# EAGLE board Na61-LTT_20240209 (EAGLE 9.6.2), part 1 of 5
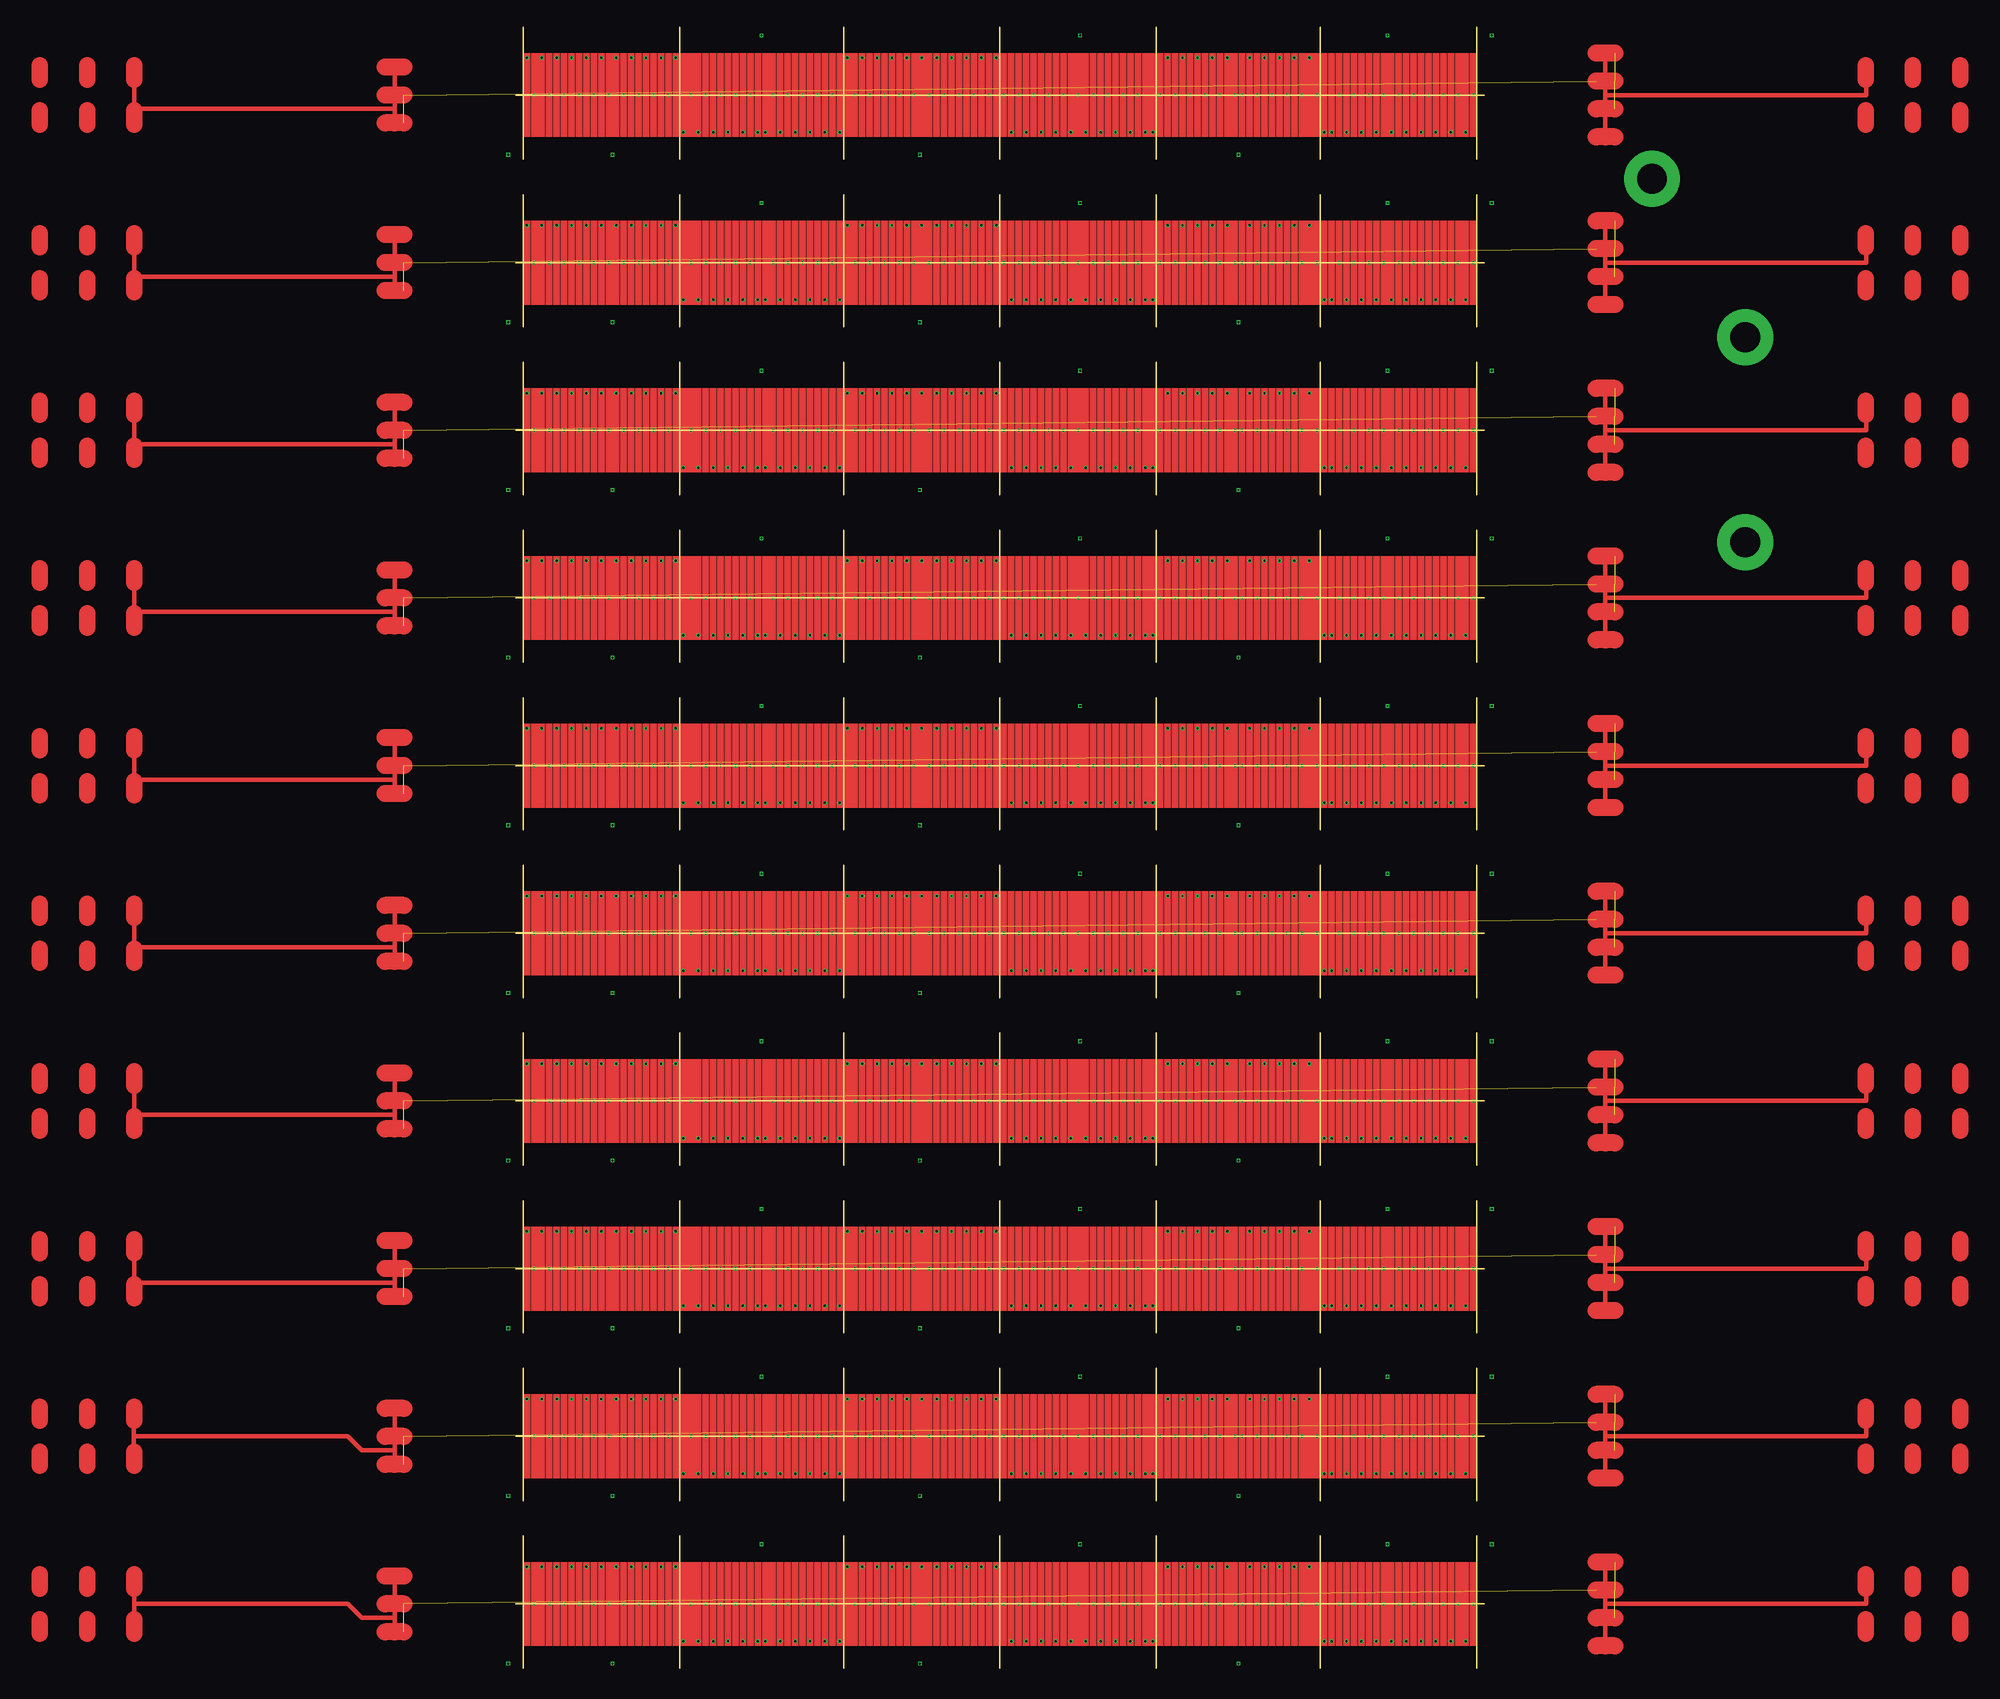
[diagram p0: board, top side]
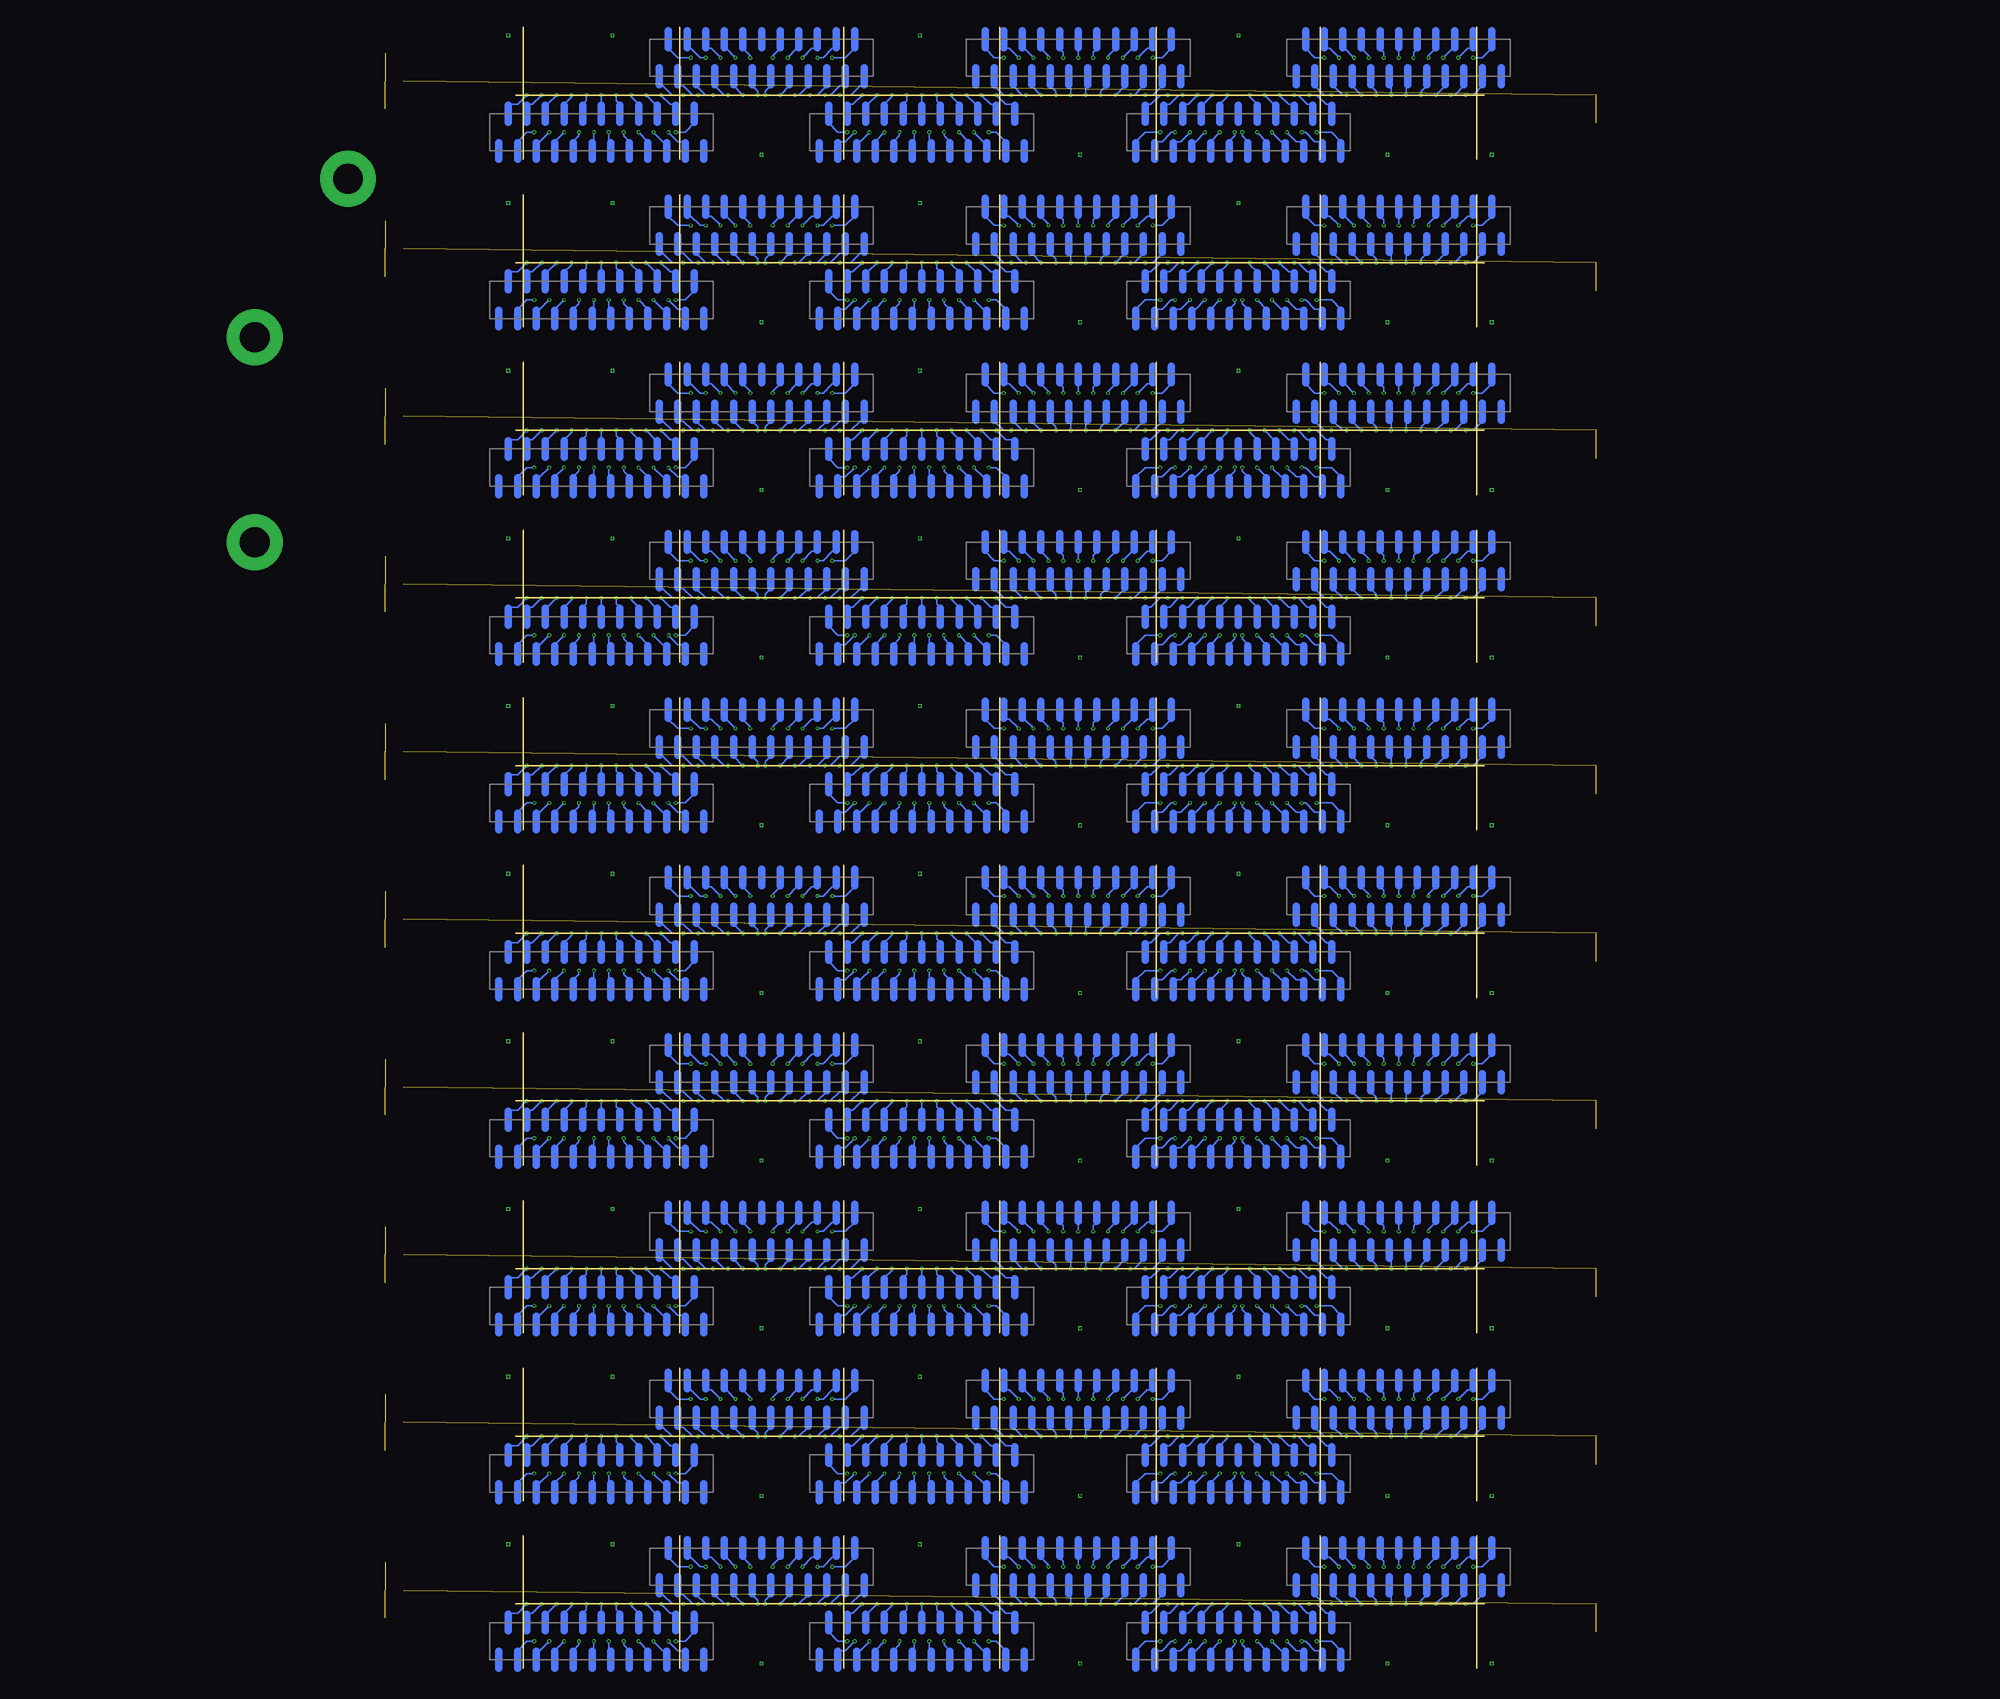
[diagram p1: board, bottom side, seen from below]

Size 104 x 176.2 mm. Coordinates in mm from the lower left corner, seen from the top.
Outline: 80 segments
Copper layers (1*16): Top 0.035mm / dielectric 1.5mm / Bottom 0.035mm
Design rules "default *": minimum track width 6mil, minimum drill 0.2mm, track to track 6mil, track to pad 6mil, pad to pad 6mil, via to via 6mil, smd to smd 6mil, copper to edge 40mil, drill to drill 6mil, minimum pad ring 8mil, minimum via ring 4mil, stop-mask expansion 4mil, vias tented up to drill 0mil, thermal gap 10mil

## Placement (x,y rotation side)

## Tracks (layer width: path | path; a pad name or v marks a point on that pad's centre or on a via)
S$1
  Bottom 0.8: 63.4,1.8 63.4,0
S$2
  Bottom 0.8: 62.4,4 62.4,5.8
S$3
  Bottom 0.8: 59.4,1.8 59.4,0
S$4
  Bottom 0.8: 56.4,4 56.4,5.8
S$5
  Bottom 0.8: 53.4,1.8 53.4,0
S$6
  Bottom 0.8: 52.4,4 52.4,5.8
S$7
  Bottom 0.8: 49.4,1.8 49.4,0
S$8
  Bottom 0.8: 50.4,4 50.4,5.8
S$9
  Bottom 0.8: 71.4,1.8 71.4,0
S$10
  Bottom 0.8: 70.4,4 70.4,5.8
S$11
  Bottom 0.8: 67.4,1.8 67.4,0
S$12
  Bottom 0.8: 66.4,4 66.4,5.8
S$13
  Bottom 0.8: 68.4,4 68.4,5.8
S$14
  Bottom 0.8: 69.4,1.8 69.4,0
S$15
  Bottom 0.8: 65.4,1.8 65.4,0
S$16
  Bottom 0.8: 64.4,4 64.4,5.8
S$17
  Bottom 0.8: 60.4,4 60.4,5.8
S$18
  Bottom 0.8: 61.4,1.8 61.4,0
S$19
  Bottom 0.8: 57.4,1.8 57.4,0
S$20
  Bottom 0.8: 58.4,4 58.4,5.8
S$21
  Bottom 0.8: 54.4,4 54.4,5.8
S$22
  Bottom 0.8: 55.4,1.8 55.4,0
S$23
  Bottom 0.8: 51.4,1.8 51.4,0
S$24
  Bottom 0.8: 44.6,9.8 44.6,8
S$25
  Bottom 0.8: 46.6,9.8 46.6,8
S$26
  Bottom 0.8: 43.6,12 43.6,13.8
S$27
  Bottom 0.8: 45.6,12 45.6,13.8
S$28
  Bottom 0.8: 40.6,9.8 40.6,8
S$29
  Bottom 0.8: 42.6,9.8 42.6,8
S$30
  Bottom 0.8: 41.6,12 41.6,13.8
S$31
  Bottom 0.8: 39.6,12 39.6,13.8
S$32
  Bottom 0.8: 38.6,9.8 38.6,8
S$33
  Bottom 0.8: 36.6,9.8 36.6,8
S$34
  Bottom 0.8: 37.6,12 37.6,13.8
S$35
  Bottom 0.8: 35.6,12 35.6,13.8
S$36
  Bottom 0.8: 34.6,9.8 34.6,8
S$37
  Bottom 0.8: 32.6,9.8 32.6,8
S$38
  Bottom 0.8: 33.6,12 33.6,13.8
S$39
  Bottom 0.8: 52.6,9.8 52.6,8
S$40
  Bottom 0.8: 54.6,9.8 54.6,8
S$41
  Bottom 0.8: 51.6,12 51.6,13.8
S$42
  Bottom 0.8: 53.6,12 53.6,13.8
S$43
  Bottom 0.8: 48.6,9.8 48.6,8
S$44
  Bottom 0.8: 50.6,9.8 50.6,8
S$45
  Bottom 0.8: 47.6,12 47.6,13.8
S$46
  Bottom 0.8: 49.6,12 49.6,13.8
S$47
  Bottom 0.8: 27.4,1.8 27.4,0
S$48
  Bottom 0.8: 29.4,1.8 29.4,0
S$49
  Bottom 0.8: 26.4,4 26.4,5.8
S$50
  Bottom 0.8: 28.4,4 28.4,5.8
S$51
  Bottom 0.8: 23.4,1.8 23.4,0
S$52
  Bottom 0.8: 25.4,1.8 25.4,0
S$53
  Bottom 0.8: 24.4,4 24.4,5.8
S$54
  Bottom 0.8: 22.4,4 22.4,5.8
S$55
  Bottom 0.8: 21.4,1.8 21.4,0
S$56
  Bottom 0.8: 19.4,1.8 19.4,0
S$57
  Bottom 0.8: 20.4,4 20.4,5.8
S$58
  Bottom 0.8: 18.4,4 18.4,5.8
S$59
  Bottom 0.8: 17.4,1.8 17.4,0
S$60
  Bottom 0.8: 15.4,1.8 15.4,0
S$61
  Bottom 0.8: 16.4,4 16.4,5.8
S$62
  Bottom 0.8: 35.4,1.8 35.4,0
S$63
  Bottom 0.8: 37.4,1.8 37.4,0
S$64
  Bottom 0.8: 34.4,4 34.4,5.8
S$65
  Bottom 0.8: 36.4,4 36.4,5.8
S$66
  Bottom 0.8: 31.4,1.8 31.4,0
S$67
  Bottom 0.8: 33.4,1.8 33.4,0
S$68
  Bottom 0.8: 30.4,4 30.4,5.8
S$69
  Bottom 0.8: 32.4,4 32.4,5.8
S$70
  Bottom 0.8: 78.6,9.8 78.6,8
S$71
  Bottom 0.8: 80.6,9.8 80.6,8
S$72
  Bottom 0.8: 77.6,12 77.6,13.8
S$73
  Bottom 0.8: 79.6,12 79.6,13.8
S$74
  Bottom 0.8: 74.6,9.8 74.6,8
S$75
  Bottom 0.8: 76.6,9.8 76.6,8
S$76
  Bottom 0.8: 75.6,12 75.6,13.8
S$77
  Bottom 0.8: 73.6,12 73.6,13.8
S$78
  Bottom 0.8: 72.6,9.8 72.6,8
S$79
  Bottom 0.8: 70.6,9.8 70.6,8
S$80
  Bottom 0.8: 71.6,12 71.6,13.8
S$81
  Bottom 0.8: 69.6,12 69.6,13.8
S$82
  Bottom 0.8: 68.6,9.8 68.6,8
S$83
  Bottom 0.8: 66.6,9.8 66.6,8
S$84
  Bottom 0.8: 67.6,12 67.6,13.8
S$85
  Bottom 0.8: 86.6,9.8 86.6,8
S$86
  Bottom 0.8: 88.6,9.8 88.6,8
S$87
  Bottom 0.8: 85.6,12 85.6,13.8
S$88
  Bottom 0.8: 87.6,12 87.6,13.8
S$89
  Bottom 0.8: 82.6,9.8 82.6,8
S$90
  Bottom 0.8: 84.6,9.8 84.6,8
S$91
  Bottom 0.8: 81.6,12 81.6,13.8
S$92
  Bottom 0.8: 83.6,12 83.6,13.8
S$93
  Bottom 0.8: 10.2,9.8 10.2,8
S$94
  Bottom 0.8: 12.2,9.8 12.2,8
S$95
  Bottom 0.8: 9.2,12 9.2,13.8
S$96
  Bottom 0.8: 11.2,12 11.2,13.8
S$97
  Bottom 0.8: 6.2,9.8 6.2,8
S$98
  Bottom 0.8: 8.2,9.8 8.2,8
S$99
  Bottom 0.8: 7.2,12 7.2,13.8
S$100
  Bottom 0.8: 5.2,12 5.2,13.8
S$101
  Bottom 0.8: 4.2,9.8 4.2,8
S$102
  Bottom 0.8: 2.2,9.8 2.2,8
S$103
  Bottom 0.8: 3.2,12 3.2,13.8
S$104
  Bottom 0.8: 1.2,12 1.2,13.8
S$105
  Bottom 0.8: 0.2,9.8 0.2,8
S$106
  Bottom 0.8: -1.8,9.8 -1.8,8
S$107
  Bottom 0.8: -0.8,12 -0.8,13.8
S$108
  Bottom 0.8: 18.2,9.8 18.2,8
S$109
  Bottom 0.8: 20.2,9.8 20.2,8
S$110
  Bottom 0.8: 17.2,12 17.2,13.8
S$111
  Bottom 0.8: 19.2,12 19.2,13.8
S$112
  Bottom 0.8: 14.2,9.8 14.2,8
S$113
  Bottom 0.8: 16.2,9.8 16.2,8
S$114
  Bottom 0.8: 13.2,12 13.2,13.8
S$115
  Bottom 0.8: 15.2,12 15.2,13.8
S$116
  Bottom 0.8: 95.8,1.8 95.8,0
S$117
  Bottom 0.8: 97.8,1.8 97.8,0
S$118
  Bottom 0.8: 94.8,4 94.8,5.8
S$119
  Bottom 0.8: 96.8,4 96.8,5.8
S$120
  Bottom 0.8: 91.8,1.8 91.8,0
S$121
  Bottom 0.8: 93.8,1.8 93.8,0
S$122
  Bottom 0.8: 92.8,4 92.8,5.8
S$123
  Bottom 0.8: 90.8,4 90.8,5.8
S$124
  Bottom 0.8: 89.8,1.8 89.8,0
S$125
  Bottom 0.8: 87.8,1.8 87.8,0
S$126
  Bottom 0.8: 88.8,4 88.8,5.8
S$127
  Bottom 0.8: 86.8,4 86.8,5.8
S$128
  Bottom 0.8: 85.8,1.8 85.8,0
S$129
  Bottom 0.8: 83.8,1.8 83.8,0
S$130
  Bottom 0.8: 84.8,4 84.8,5.8
S$131
  Bottom 0.8: 103.8,1.8 103.8,0
S$132
  Bottom 0.8: 105.8,1.8 105.8,0
S$133
  Bottom 0.8: 102.8,4 102.8,5.8
S$134
  Bottom 0.8: 104.8,4 104.8,5.8
S$135
  Bottom 0.8: 99.8,1.8 99.8,0
S$136
  Bottom 0.8: 101.8,1.8 101.8,0
S$137
  Bottom 0.8: 98.8,4 98.8,5.8
S$138
  Bottom 0.8: 100.8,4 100.8,5.8
S$139  (4 unrouted)
  Top 0.508: -13,9.9 -13,5.4 | -13,5.4 -13,3.9 | -13,5.4 -16.5,5.4 -18,6.9 -40.5,6.9 -40.92,6.9 -40.92,5.4 -40.92,7.9 | 117,11.4 117,6.9 | 117,6.9 117,2.4 | 117,6.9 145,6.9 145,8.9
  Top 1.8: -12,6.9 -14,6.9 | -12,9.9 -13,9.9 -14,9.9 | -12,3.9 -13,3.9 -14,3.9 | 118,8.4 116,8.4 | 118,11.4 117,11.4 116,11.4 | 118,5.4 116,5.4 | 118,2.4 117,2.4 116,2.4
S$140
  Top 1.778: -51.08,8.55 -51.08,10.07
S$141  (via drill 0.2)
  other vias: 26.4,13.3
S$142
  Top 1.778: -46,8.55 -46,10.07
S$143
  Top 1.778: -40.92,8.55 -40.92,10.07
S$144
  Top 1.778: 144.92,3.73 144.92,5.25
S$145
  Bottom 0.8: 61.4,19.8 61.4,18
S$146
  Top 1.778: 144.92,8.55 144.92,10.07
S$147
  Top 1.778: 150,3.73 150,5.25
S$148
  Top 1.778: 150,8.55 150,10.07
S$149
  Top 1.778: 155.08,3.73 155.08,5.25
S$150
  Top 1.778: 155.08,8.55 155.08,10.07
S$151  (via drill 0.2)
  other vias: 43.4,0.5
S$152  (via drill 0.2)
  other vias: 60.6,13.3
S$153  (via drill 0.2)
  other vias: 77.6,0.5
S$154  (via drill 0.2)
  other vias: 93.6,13.3
S$155  (via drill 0.2)
  other vias: 104.8,13.3
S$156  (via drill 0.2)
  other vias: 10.4,0.5
S$157  (via drill 0.2)
  other vias: -0.8,0.5
S$158
  Bottom 0.8: 63.4,19.8 63.4,18
S$159
  Bottom 0.8: 60.4,22 60.4,23.8
S$160
  Bottom 0.8: 62.4,22 62.4,23.8
S$161
  Bottom 0.8: 57.4,19.8 57.4,18
S$162  (via drill 0.2)
  other vias: 1.2,10.9
S$163  (via drill 0.2)
  other vias: 2.8,10.9
S$164  (via drill 0.2)
  other vias: 4.4,10.9
S$165  (via drill 0.2)
  other vias: 6,10.9
S$166  (via drill 0.2)
  other vias: 7.6,10.9
S$167  (via drill 0.2)
  other vias: 9.2,10.9
S$168  (via drill 0.2)
  other vias: 10.8,10.9
S$169  (via drill 0.2)
  other vias: 12.4,10.9
S$170  (via drill 0.2)
  other vias: 14,10.9
S$171  (via drill 0.2)
  other vias: 15.6,10.9
S$172  (via drill 0.2)
  other vias: 17.2,10.9
S$173  (via drill 0.2)
  other vias: 2,6.9
S$174  (via drill 0.2)
  other vias: 3.6,6.9
S$175  (via drill 0.2)
  other vias: 5.2,6.9
S$176  (via drill 0.2)
  other vias: 6.8,6.9
S$177  (via drill 0.2)
  other vias: 8.4,6.9
S$178  (via drill 0.2)
  other vias: 10,6.9
S$179  (via drill 0.2)
  other vias: 11.6,6.9
S$180  (via drill 0.2)
  other vias: 13.2,6.9
S$181  (via drill 0.2)
  other vias: 14.8,6.9
S$182  (via drill 0.2)
  other vias: 16.4,6.9
S$183  (via drill 0.2)
  other vias: 18,2.9
S$184  (via drill 0.2)
  other vias: 19.6,2.9
S$185  (via drill 0.2)
  other vias: 21.2,2.9
S$186  (via drill 0.2)
  other vias: 22.8,2.9
S$187  (via drill 0.2)
  other vias: 24.4,2.9
S$188  (via drill 0.2)
  other vias: 18.8,6.9
S$189  (via drill 0.2)
  other vias: 20.4,6.9
S$190  (via drill 0.2)
  other vias: 22,6.9
S$191  (via drill 0.2)
  other vias: 23.6,6.9
S$192  (via drill 0.2)
  other vias: 25.2,6.9
S$193  (via drill 0.2)
  other vias: 26,2.9
S$194  (via drill 0.2)
  other vias: 51.6,10.9
S$195  (via drill 0.2)
  other vias: 50,10.9
S$196  (via drill 0.2)
  other vias: 48.4,10.9
S$197  (via drill 0.2)
  other vias: 46.8,10.9
S$198  (via drill 0.2)
  other vias: 45.2,10.9
S$199  (via drill 0.2)
  other vias: 43.6,10.9
S$200  (via drill 0.2)
  other vias: 42,10.9
S$201  (via drill 0.2)
  other vias: 40.4,10.9
S$202  (via drill 0.2)
  other vias: 38.8,10.9
S$203  (via drill 0.2)
  other vias: 37.2,10.9
S$204  (via drill 0.2)
  other vias: 35.6,10.9
S$205  (via drill 0.2)
  other vias: 50.8,6.9
S$206  (via drill 0.2)
  other vias: 49.2,6.9
S$207  (via drill 0.2)
  other vias: 47.6,6.9
S$208  (via drill 0.2)
  other vias: 46,6.9
S$209  (via drill 0.2)
  other vias: 44.4,6.9
S$210  (via drill 0.2)
  other vias: 42.8,6.9
S$211  (via drill 0.2)
  other vias: 41.2,6.9
S$212  (via drill 0.2)
  other vias: 39.6,6.9
S$213  (via drill 0.2)
  other vias: 38,6.9
S$214  (via drill 0.2)
  other vias: 36.4,6.9
S$215  (via drill 0.2)
  other vias: 34.8,2.9
S$216  (via drill 0.2)
  other vias: 33.2,2.9
S$217  (via drill 0.2)
  other vias: 31.6,2.9
S$218  (via drill 0.2)
  other vias: 30,2.9
S$219  (via drill 0.2)
  other vias: 28.4,2.9
S$220  (via drill 0.2)
  other vias: 34,6.9
S$221  (via drill 0.2)
  other vias: 32.4,6.9
S$222  (via drill 0.2)
  other vias: 30.8,6.9
S$223  (via drill 0.2)
  other vias: 29.2,6.9
S$224  (via drill 0.2)
  other vias: 27.6,6.9
S$225  (via drill 0.2)
  other vias: 26.8,2.9
S$226  (via drill 0.2)
  other vias: 52.4,6.9
S$227  (via drill 0.2)
  other vias: 54,6.9
S$228  (via drill 0.2)
  other vias: 55.6,6.9
S$229  (via drill 0.2)
  other vias: 57.2,6.9
S$230  (via drill 0.2)
  other vias: 58.8,6.9
S$231  (via drill 0.2)
  other vias: 60.4,6.9
S$232  (via drill 0.2)
  other vias: 62,6.9
S$233  (via drill 0.2)
  other vias: 63.6,6.9
S$234  (via drill 0.2)
  other vias: 65.2,6.9
S$235  (via drill 0.2)
  other vias: 66.8,6.9
S$236  (via drill 0.2)
  other vias: 68.4,2.9
S$237  (via drill 0.2)
  other vias: 53.2,2.9
S$238  (via drill 0.2)
  other vias: 54.8,2.9
S$239  (via drill 0.2)
  other vias: 56.4,2.9
S$240  (via drill 0.2)
  other vias: 58,2.9
S$241  (via drill 0.2)
  other vias: 59.6,2.9
S$242  (via drill 0.2)
  other vias: 61.2,2.9
S$243  (via drill 0.2)
  other vias: 62.8,2.9
S$244  (via drill 0.2)
  other vias: 64.4,2.9
S$245  (via drill 0.2)
  other vias: 66,2.9
S$246  (via drill 0.2)
  other vias: 67.6,2.9
S$247  (via drill 0.2)
  other vias: 69.2,6.9
S$248  (via drill 0.2)
  other vias: 70.8,6.9
S$249  (via drill 0.2)
  other vias: 72.4,6.9
S$250  (via drill 0.2)
  other vias: 70,10.9
S$251  (via drill 0.2)
  other vias: 71.6,10.9
S$252  (via drill 0.2)
  other vias: 73.2,10.9
S$253  (via drill 0.2)
  other vias: 74,6.9
S$254  (via drill 0.2)
  other vias: 74.8,10.9
S$255  (via drill 0.2)
  other vias: 75.6,6.9
S$256  (via drill 0.2)
  other vias: 76.4,10.9
S$257  (via drill 0.2)
  other vias: 77.2,6.9
S$258  (via drill 0.2)
  other vias: 102.8,6.9
S$259  (via drill 0.2)
  other vias: 101.2,6.9
S$260  (via drill 0.2)
  other vias: 99.6,6.9
S$261  (via drill 0.2)
  other vias: 98,6.9
S$262  (via drill 0.2)
  other vias: 96.4,6.9
S$263  (via drill 0.2)
  other vias: 94.8,6.9
S$264  (via drill 0.2)
  other vias: 93.2,6.9
S$265  (via drill 0.2)
  other vias: 91.6,6.9
S$266  (via drill 0.2)
  other vias: 90,6.9
S$267  (via drill 0.2)
  other vias: 88.4,6.9
S$268  (via drill 0.2)
  other vias: 86.8,2.9
S$269  (via drill 0.2)
  other vias: 102,2.9
S$270  (via drill 0.2)
  other vias: 100.4,2.9
S$271  (via drill 0.2)
  other vias: 98.8,2.9
S$272  (via drill 0.2)
  other vias: 97.2,2.9
S$273  (via drill 0.2)
  other vias: 95.6,2.9
S$274  (via drill 0.2)
  other vias: 94,2.9
S$275  (via drill 0.2)
  other vias: 92.4,2.9
S$276  (via drill 0.2)
  other vias: 90.8,2.9
S$277  (via drill 0.2)
  other vias: 89.2,2.9
S$278  (via drill 0.2)
  other vias: 87.6,2.9
S$279  (via drill 0.2)
  other vias: 86,6.9
S$280  (via drill 0.2)
  other vias: 84.4,6.9
S$281  (via drill 0.2)
  other vias: 82.8,6.9
S$282  (via drill 0.2)
  other vias: 85.2,10.9
S$283  (via drill 0.2)
  other vias: 83.6,10.9
S$284  (via drill 0.2)
  other vias: 82,10.9
S$285  (via drill 0.2)
  other vias: 81.2,6.9
S$286  (via drill 0.2)
  other vias: 80.4,10.9
S$287  (via drill 0.2)
  other vias: 79.6,6.9
S$288  (via drill 0.2)
  other vias: 78.8,10.9
S$289  (via drill 0.2)
  other vias: 78,6.9
S$290
  Bottom 0.152: -0.8,11.9 0.2,10.9
S$291
  Bottom 0.152: 0.2,10.9 1.2,10.9
S$292
  Bottom 0.152: 1.2,11.9 1.8,11.9
S$293
  Bottom 0.152: 1.8,11.9 2.8,10.9
S$294
  Bottom 0.152: 3.2,11.9 3.4,11.9
S$295
  Bottom 0.152: 3.4,11.9 4.4,10.9
S$296
  Bottom 0.152: 5.2,11.9 6,11.1
S$297
  Bottom 0.152: 6,11.1 6,10.9
S$298
  Bottom 0.152: 7.2,11.9 7.6,11.5
S$299
  Bottom 0.152: 7.6,11.5 7.6,10.9
S$300
  Bottom 0.152: 9.2,11.9 9.2,10.9
S$301
  Bottom 0.152: 11.2,11.9 10.8,11.5
S$302
  Bottom 0.152: 10.8,11.5 10.8,10.9
S$303
  Bottom 0.152: 13.2,11.9 12.4,11.1
S$304
  Bottom 0.152: 12.4,11.1 12.4,10.9
S$305
  Bottom 0.152: 15.2,11.9 15,11.9
S$306
  Bottom 0.152: 15,11.9 14,10.9
S$307
  Bottom 0.152: 17.2,11.9 16.6,11.9
S$308
  Bottom 0.152: 16.6,11.9 15.6,10.9
S$309
  Bottom 0.152: 19.2,11.9 18.2,10.9
S$310
  Bottom 0.152: 18.2,10.9 17.2,10.9
S$311
  Bottom 0.152: 0.2,7.9 1.2,6.9
S$312
  Bottom 0.152: 1.2,6.9 2,6.9
S$313
  Bottom 0.152: 2.2,7.9 3.2,6.9
S$314
  Bottom 0.152: 3.2,6.9 3.6,6.9
S$315
  Bottom 0.152: 4.2,7.9 5.2,6.9
S$316
  Bottom 0.152: 6.2,7.9 6.8,7.3
S$317
  Bottom 0.152: 6.8,7.3 6.8,6.9
S$318
  Bottom 0.152: 8.2,7.9 8.4,7.7
S$319
  Bottom 0.152: 8.4,7.7 8.4,6.9
S$320
  Bottom 0.152: 10.2,7.9 10,7.7
S$321
  Bottom 0.152: 10,7.7 10,6.9
S$322
  Bottom 0.152: 12.2,7.9 11.6,7.3
S$323
  Bottom 0.152: 11.6,7.3 11.6,6.9
S$324
  Bottom 0.152: 14.2,7.9 13.2,6.9
S$325
  Bottom 0.152: 16.2,7.9 15.2,6.9
S$326
  Bottom 0.152: 15.2,6.9 14.8,6.9
S$327
  Bottom 0.152: 18.2,7.9 17.2,6.9
S$328
  Bottom 0.152: 17.2,6.9 16.4,6.9
S$329
  Bottom 0.152: 15.4,1.9 16.4,2.9
S$330
  Bottom 0.152: 16.4,2.9 18,2.9
S$331
  Bottom 0.152: 17.4,1.9 18.2,1.9
S$332
  Bottom 0.152: 18.2,1.9 19.2,2.9
S$333
  Bottom 0.152: 19.2,2.9 19.6,2.9
S$334
  Bottom 0.152: 19.4,1.9 20.2,1.9
S$335
  Bottom 0.152: 20.2,1.9 21.2,2.9
S$336
  Bottom 0.152: 21.4,1.9 21.8,1.9
S$337
  Bottom 0.152: 21.8,1.9 22.8,2.9
S$338
  Bottom 0.152: 23.4,1.9 24.4,2.9
S$339
  Bottom 0.152: 25.4,1.9 26,2.5
S$340
  Bottom 0.152: 26,2.5 26,2.9
S$341
  Bottom 0.152: 16.4,5.9 17,5.9
S$342
  Bottom 0.152: 17,5.9 18,6.9
S$343
  Bottom 0.152: 18,6.9 18.8,6.9
S$344
  Bottom 0.152: 18.4,5.9 19,5.9
S$345
  Bottom 0.152: 19,5.9 20,6.9
S$346
  Bottom 0.152: 20,6.9 20.4,6.9
S$347
  Bottom 0.152: 20.4,5.9 21,5.9
S$348
  Bottom 0.152: 21,5.9 22,6.9
S$349
  Bottom 0.152: 22.4,5.9 22.6,5.9
S$350
  Bottom 0.152: 22.6,5.9 23.6,6.9
S$351
  Bottom 0.152: 24.4,5.9 25.2,6.7
S$352
  Bottom 0.152: 25.2,6.7 25.2,6.9
S$353
  Bottom 0.152: 53.6,11.9 52.6,10.9
S$354
  Bottom 0.152: 52.6,10.9 51.6,10.9
S$355
  Bottom 0.152: 51.6,11.9 51,11.9
S$356
  Bottom 0.152: 51,11.9 50,10.9
S$357
  Bottom 0.152: 49.6,11.9 49.4,11.9
S$358
  Bottom 0.152: 49.4,11.9 48.4,10.9
S$359
  Bottom 0.152: 47.6,11.9 46.8,11.1
S$360
  Bottom 0.152: 46.8,11.1 46.8,10.9
S$361
  Bottom 0.152: 45.6,11.9 45.2,11.5
S$362
  Bottom 0.152: 45.2,11.5 45.2,10.9
S$363
  Bottom 0.152: 43.6,11.9 43.6,10.9
S$364
  Bottom 0.152: 41.6,11.9 42,11.5
S$365
  Bottom 0.152: 42,11.5 42,10.9
S$366
  Bottom 0.152: 39.6,11.9 40.4,11.1
S$367
  Bottom 0.152: 40.4,11.1 40.4,10.9
S$368
  Bottom 0.152: 37.6,11.9 37.8,11.9
S$369
  Bottom 0.152: 37.8,11.9 38.8,10.9
S$370
  Bottom 0.152: 35.6,11.9 36.2,11.9
S$371
  Bottom 0.152: 36.2,11.9 37.2,10.9
S$372
  Bottom 0.152: 33.6,11.9 34.6,10.9
S$373
  Bottom 0.152: 34.6,10.9 35.6,10.9
S$374
  Bottom 0.152: 52.6,7.9 51.6,6.9
S$375
  Bottom 0.152: 51.6,6.9 50.8,6.9
S$376
  Bottom 0.152: 50.6,7.9 49.6,6.9
S$377
  Bottom 0.152: 49.6,6.9 49.2,6.9
S$378
  Bottom 0.152: 48.6,7.9 47.6,6.9
S$379
  Bottom 0.152: 46.6,7.9 46,7.3
S$380
  Bottom 0.152: 46,7.3 46,6.9
S$381
  Bottom 0.152: 44.6,7.9 44.4,7.7
S$382
  Bottom 0.152: 44.4,7.7 44.4,6.9
S$383
  Bottom 0.152: 42.6,7.9 42.8,7.7
S$384
  Bottom 0.152: 42.8,7.7 42.8,6.9
S$385
  Bottom 0.152: 40.6,7.9 41.2,7.3
S$386
  Bottom 0.152: 41.2,7.3 41.2,6.9
S$387
  Bottom 0.152: 38.6,7.9 39.6,6.9
S$388
  Bottom 0.152: 36.6,7.9 37.6,6.9
S$389
  Bottom 0.152: 37.6,6.9 38,6.9
S$390
  Bottom 0.152: 34.6,7.9 35.6,6.9
S$391
  Bottom 0.152: 35.6,6.9 36.4,6.9
S$392
  Bottom 0.152: 37.4,1.9 36.4,2.9
S$393
  Bottom 0.152: 36.4,2.9 34.8,2.9
S$394
  Bottom 0.152: 35.4,1.9 34.6,1.9
S$395
  Bottom 0.152: 34.6,1.9 33.6,2.9
S$396
  Bottom 0.152: 33.6,2.9 33.2,2.9
S$397
  Bottom 0.152: 33.4,1.9 32.6,1.9
S$398
  Bottom 0.152: 32.6,1.9 31.6,2.9
S$399
  Bottom 0.152: 31.4,1.9 31,1.9
S$400
  Bottom 0.152: 31,1.9 30,2.9
S$401
  Bottom 0.152: 29.4,1.9 28.4,2.9
S$402
  Bottom 0.152: 27.4,1.9 26.8,2.5
S$403
  Bottom 0.152: 26.8,2.5 26.8,2.9
S$404
  Bottom 0.152: 36.4,5.9 35.8,5.9
S$405
  Bottom 0.152: 35.8,5.9 34.8,6.9
S$406
  Bottom 0.152: 34.8,6.9 34,6.9
S$407
  Bottom 0.152: 34.4,5.9 33.8,5.9
S$408
  Bottom 0.152: 33.8,5.9 32.8,6.9
S$409
  Bottom 0.152: 32.8,6.9 32.4,6.9
S$410
  Bottom 0.152: 32.4,5.9 31.8,5.9
S$411
  Bottom 0.152: 31.8,5.9 30.8,6.9
S$412
  Bottom 0.152: 30.4,5.9 30.2,5.9
S$413
  Bottom 0.152: 30.2,5.9 29.2,6.9
S$414
  Bottom 0.152: 28.4,5.9 27.6,6.7
S$415
  Bottom 0.152: 27.6,6.7 27.6,6.9
S$416
  Bottom 0.152: 52.4,5.9 53,5.9
S$417
  Bottom 0.152: 53,5.9 54,6.9
S$418
  Bottom 0.152: 54.4,5.9 54.6,5.9
S$419
  Bottom 0.152: 54.6,5.9 55.6,6.9
S$420
  Bottom 0.152: 56.4,5.9 57.2,6.7
S$421
  Bottom 0.152: 57.2,6.7 57.2,6.9
S$422
  Bottom 0.152: 58.4,5.9 58.8,6.3
S$423
  Bottom 0.152: 58.8,6.3 58.8,6.9
S$424
  Bottom 0.152: 60.4,5.9 60.4,6.9
S$425
  Bottom 0.152: 50.4,5.9 51.4,5.9
S$426
  Bottom 0.152: 51.4,5.9 52.4,6.9
S$427
  Bottom 0.152: 51.4,1.9 52.4,2.9
S$428
  Bottom 0.152: 52.4,2.9 53.2,2.9
S$429
  Bottom 0.152: 53.4,1.9 53.8,1.9
S$430
  Bottom 0.152: 53.8,1.9 54.8,2.9
S$431
  Bottom 0.152: 55.4,1.9 56.4,2.9
S$432
  Bottom 0.152: 57.4,1.9 58,2.5
S$433
  Bottom 0.152: 58,2.5 58,2.9
S$434
  Bottom 0.152: 59.4,1.9 59.6,2.1
S$435
  Bottom 0.152: 59.6,2.1 59.6,2.9
S$436
  Bottom 0.152: 61.4,1.9 61.2,2.1
S$437
  Bottom 0.152: 61.2,2.1 61.2,2.9
S$438
  Bottom 0.152: 63.4,1.9 62.8,2.5
S$439
  Bottom 0.152: 62.8,2.5 62.8,2.9
S$440
  Bottom 0.152: 65.4,1.9 64.4,2.9
S$441
  Bottom 0.152: 67.4,1.9 67,1.9
S$442
  Bottom 0.152: 67,1.9 66,2.9
S$443
  Bottom 0.152: 69.4,1.9 68.6,1.9
S$444
  Bottom 0.152: 68.6,1.9 67.6,2.9
S$445
  Bottom 0.152: 62.4,5.9 62,6.3
S$446
  Bottom 0.152: 62,6.3 62,6.9
S$447
  Bottom 0.152: 64.4,5.9 63.6,6.7
S$448
  Bottom 0.152: 63.6,6.7 63.6,6.9
S$449
  Bottom 0.152: 66.4,5.9 66.2,5.9
S$450
  Bottom 0.152: 66.2,5.9 65.2,6.9
S$451
  Bottom 0.152: 68.4,5.9 67.8,5.9
S$452
  Bottom 0.152: 67.8,5.9 66.8,6.9
S$453
  Bottom 0.152: 70.4,3.9 69.4,2.9
S$454
  Bottom 0.152: 69.4,2.9 68.4,2.9
S$455
  Bottom 0.152: 68.6,7.9 69.2,7.9
S$456
  Bottom 0.152: 69.2,7.9 70.2,6.9
S$457
  Bottom 0.152: 70.2,6.9 70.8,6.9
S$458
  Bottom 0.152: 70.6,7.9 71.6,6.9
S$459
  Bottom 0.152: 71.6,6.9 72.4,6.9
S$460
  Bottom 0.152: 72.6,7.9 73.6,6.9
S$461
  Bottom 0.152: 73.6,6.9 74,6.9
S$462
  Bottom 0.152: 74.6,7.9 75.6,6.9
S$463
  Bottom 0.152: 76.6,7.9 77.2,7.3
S$464
  Bottom 0.152: 77.2,7.3 77.2,6.9
S$465
  Bottom 0.152: 67.6,11.9 68.6,10.9
S$466
  Bottom 0.152: 68.6,10.9 70,10.9
S$467
  Bottom 0.152: 69.6,11.9 70,11.9
S$468
  Bottom 0.152: 70,11.9 71,10.9
S$469
  Bottom 0.152: 71,10.9 71.6,10.9
S$470
  Bottom 0.152: 71.6,11.9 72.2,11.9
S$471
  Bottom 0.152: 72.2,11.9 73.2,10.9
S$472
  Bottom 0.152: 73.6,11.9 73.8,11.9
S$473
  Bottom 0.152: 73.8,11.9 74.8,10.9
S$474
  Bottom 0.152: 75.6,11.9 76.4,11.1
S$475
  Bottom 0.152: 76.4,11.1 76.4,10.9
S$476
  Bottom 0.152: 69.2,6.9 68,6.9
S$477
  Bottom 0.152: 68,6.9 67,7.9
S$478
  Bottom 0.152: 67,7.9 66.6,7.9
S$479
  Bottom 0.152: 102.8,5.9 102.2,5.9
S$480
  Bottom 0.152: 102.2,5.9 101.2,6.9
S$481
  Bottom 0.152: 100.8,5.9 100.6,5.9
S$482
  Bottom 0.152: 100.6,5.9 99.6,6.9
S$483
  Bottom 0.152: 98.8,5.9 98,6.7
S$484
  Bottom 0.152: 98,6.7 98,6.9
S$485
  Bottom 0.152: 96.8,5.9 96.4,6.3
S$486
  Bottom 0.152: 96.4,6.3 96.4,6.9
S$487
  Bottom 0.152: 94.8,5.9 94.8,6.9
S$488
  Bottom 0.152: 104.8,5.9 103.8,5.9
S$489
  Bottom 0.152: 103.8,5.9 102.8,6.9
S$490
  Bottom 0.152: 103.8,1.9 102.8,2.9
S$491
  Bottom 0.152: 102.8,2.9 102,2.9
S$492
  Bottom 0.152: 101.8,1.9 101.4,1.9
S$493
  Bottom 0.152: 101.4,1.9 100.4,2.9
S$494
  Bottom 0.152: 99.8,1.9 98.8,2.9
S$495
  Bottom 0.152: 97.8,1.9 97.2,2.5
S$496
  Bottom 0.152: 97.2,2.5 97.2,2.9
S$497
  Bottom 0.152: 95.8,1.9 95.6,2.1
S$498
  Bottom 0.152: 95.6,2.1 95.6,2.9
S$499
  Bottom 0.152: 93.8,1.9 94,2.1
S$500
  Bottom 0.152: 94,2.1 94,2.9
S$501
  Bottom 0.152: 91.8,1.9 92.4,2.5
S$502
  Bottom 0.152: 92.4,2.5 92.4,2.9
S$503
  Bottom 0.152: 89.8,1.9 90.8,2.9
S$504
  Bottom 0.152: 87.8,1.9 88.2,1.9
S$505
  Bottom 0.152: 88.2,1.9 89.2,2.9
S$506
  Bottom 0.152: 85.8,1.9 86.6,1.9
S$507
  Bottom 0.152: 86.6,1.9 87.6,2.9
S$508
  Bottom 0.152: 92.8,5.9 93.2,6.3
S$509
  Bottom 0.152: 93.2,6.3 93.2,6.9
S$510
  Bottom 0.152: 90.8,5.9 91.6,6.7
S$511
  Bottom 0.152: 91.6,6.7 91.6,6.9
S$512
  Bottom 0.152: 88.8,5.9 89,5.9
S$513
  Bottom 0.152: 89,5.9 90,6.9
S$514
  Bottom 0.152: 86.8,5.9 87.4,5.9
S$515
  Bottom 0.152: 87.4,5.9 88.4,6.9
S$516
  Bottom 0.152: 84.8,3.9 85.8,2.9
S$517
  Bottom 0.152: 85.8,2.9 86.8,2.9
S$518
  Bottom 0.152: 86.6,7.9 86,7.9
S$519
  Bottom 0.152: 86,7.9 85,6.9
S$520
  Bottom 0.152: 85,6.9 84.4,6.9
S$521
  Bottom 0.152: 84.6,7.9 83.6,6.9
S$522
  Bottom 0.152: 83.6,6.9 82.8,6.9
S$523
  Bottom 0.152: 82.6,7.9 81.6,6.9
S$524
  Bottom 0.152: 81.6,6.9 81.2,6.9
S$525
  Bottom 0.152: 80.6,7.9 79.6,6.9
S$526
  Bottom 0.152: 78.6,7.9 78,7.3
S$527
  Bottom 0.152: 78,7.3 78,6.9
S$528
  Bottom 0.152: 87.6,11.9 86.6,10.9
S$529
  Bottom 0.152: 86.6,10.9 85.2,10.9
S$530
  Bottom 0.152: 85.6,11.9 85.2,11.9
S$531
  Bottom 0.152: 85.2,11.9 84.2,10.9
S$532
  Bottom 0.152: 84.2,10.9 83.6,10.9
S$533
  Bottom 0.152: 83.6,11.9 83,11.9
S$534
  Bottom 0.152: 83,11.9 82,10.9
S$535
  Bottom 0.152: 81.6,11.9 81.4,11.9
S$536
  Bottom 0.152: 81.4,11.9 80.4,10.9
S$537
  Bottom 0.152: 79.6,11.9 78.8,11.1
S$538
  Bottom 0.152: 78.8,11.1 78.8,10.9
S$539
  Bottom 0.152: 86,6.9 87.2,6.9
S$540
  Bottom 0.152: 87.2,6.9 88.2,7.9
S$541
  Bottom 0.152: 88.2,7.9 88.6,7.9
S$542
  Bottom 0.8: 59.4,19.8 59.4,18
S$543
  Bottom 0.8: 58.4,22 58.4,23.8
S$544
  Bottom 0.8: 56.4,22 56.4,23.8
S$545
  Bottom 0.8: 55.4,19.8 55.4,18
S$546
  Bottom 0.8: 53.4,19.8 53.4,18
S$547
  Bottom 0.8: 54.4,22 54.4,23.8
S$548
  Bottom 0.8: 52.4,22 52.4,23.8
S$549
  Bottom 0.8: 51.4,19.8 51.4,18
S$550
  Bottom 0.8: 49.4,19.8 49.4,18
S$551
  Bottom 0.8: 50.4,22 50.4,23.8
S$552
  Bottom 0.8: 69.4,19.8 69.4,18
S$553
  Bottom 0.8: 71.4,19.8 71.4,18
S$554
  Bottom 0.8: 68.4,22 68.4,23.8
S$555
  Bottom 0.8: 70.4,22 70.4,23.8
S$556
  Bottom 0.8: 65.4,19.8 65.4,18
S$557
  Bottom 0.8: 67.4,19.8 67.4,18
S$558
  Bottom 0.8: 64.4,22 64.4,23.8
S$559
  Bottom 0.8: 66.4,22 66.4,23.8
S$560
  Bottom 0.8: 44.6,27.8 44.6,26
S$561
  Bottom 0.8: 46.6,27.8 46.6,26
S$562
  Bottom 0.8: 43.6,30 43.6,31.8
S$563
  Bottom 0.8: 45.6,30 45.6,31.8
S$564
  Bottom 0.8: 40.6,27.8 40.6,26
S$565
  Bottom 0.8: 42.6,27.8 42.6,26
S$566
  Bottom 0.8: 41.6,30 41.6,31.8
S$567
  Bottom 0.8: 39.6,30 39.6,31.8
S$568
  Bottom 0.8: 38.6,27.8 38.6,26
S$569
  Bottom 0.8: 36.6,27.8 36.6,26
S$570
  Bottom 0.8: 37.6,30 37.6,31.8
S$571
  Bottom 0.8: 35.6,30 35.6,31.8
S$572
  Bottom 0.8: 34.6,27.8 34.6,26
S$573
  Bottom 0.8: 32.6,27.8 32.6,26
S$574
  Bottom 0.8: 33.6,30 33.6,31.8
S$575
  Bottom 0.8: 52.6,27.8 52.6,26
S$576
  Bottom 0.8: 54.6,27.8 54.6,26
S$577
  Bottom 0.8: 51.6,30 51.6,31.8
S$578
  Bottom 0.8: 53.6,30 53.6,31.8
S$579
  Bottom 0.8: 48.6,27.8 48.6,26
S$580
  Bottom 0.8: 50.6,27.8 50.6,26
S$581
  Bottom 0.8: 47.6,30 47.6,31.8
S$582
  Bottom 0.8: 49.6,30 49.6,31.8
S$583
  Bottom 0.8: 27.4,19.8 27.4,18
S$584
  Bottom 0.8: 29.4,19.8 29.4,18
S$585
  Bottom 0.8: 26.4,22 26.4,23.8
S$586
  Bottom 0.8: 28.4,22 28.4,23.8
S$587
  Bottom 0.8: 23.4,19.8 23.4,18
S$588
  Bottom 0.8: 25.4,19.8 25.4,18
S$589
  Bottom 0.8: 24.4,22 24.4,23.8
S$590
  Bottom 0.8: 22.4,22 22.4,23.8
S$591
  Bottom 0.8: 21.4,19.8 21.4,18
S$592
  Bottom 0.8: 19.4,19.8 19.4,18
S$593
  Bottom 0.8: 20.4,22 20.4,23.8
S$594
  Bottom 0.8: 18.4,22 18.4,23.8
S$595
  Bottom 0.8: 17.4,19.8 17.4,18
S$596
  Bottom 0.8: 15.4,19.8 15.4,18
S$597
  Bottom 0.8: 16.4,22 16.4,23.8
S$598
  Bottom 0.8: 35.4,19.8 35.4,18
S$599
  Bottom 0.8: 37.4,19.8 37.4,18
S$600
  Bottom 0.8: 34.4,22 34.4,23.8
S$601
  Bottom 0.8: 36.4,22 36.4,23.8
S$602
  Bottom 0.8: 31.4,19.8 31.4,18
S$603
  Bottom 0.8: 33.4,19.8 33.4,18
S$604
  Bottom 0.8: 30.4,22 30.4,23.8
S$605
  Bottom 0.8: 32.4,22 32.4,23.8
S$606
  Bottom 0.8: 78.6,27.8 78.6,26
S$607
  Bottom 0.8: 80.6,27.8 80.6,26
S$608
  Bottom 0.8: 77.6,30 77.6,31.8
S$609
  Bottom 0.8: 79.6,30 79.6,31.8
S$610
  Bottom 0.8: 74.6,27.8 74.6,26
S$611
  Bottom 0.8: 76.6,27.8 76.6,26
S$612
  Bottom 0.8: 75.6,30 75.6,31.8
S$613
  Bottom 0.8: 73.6,30 73.6,31.8
S$614
  Bottom 0.8: 72.6,27.8 72.6,26
S$615
  Bottom 0.8: 70.6,27.8 70.6,26
S$616
  Bottom 0.8: 71.6,30 71.6,31.8
S$617
  Bottom 0.8: 69.6,30 69.6,31.8
S$618
  Bottom 0.8: 68.6,27.8 68.6,26
S$619
  Bottom 0.8: 66.6,27.8 66.6,26
S$620
  Bottom 0.8: 67.6,30 67.6,31.8
S$621
  Bottom 0.8: 86.6,27.8 86.6,26
S$622
  Bottom 0.8: 88.6,27.8 88.6,26
S$623
  Bottom 0.8: 85.6,30 85.6,31.8
S$624
  Bottom 0.8: 87.6,30 87.6,31.8
S$625
  Bottom 0.8: 82.6,27.8 82.6,26
S$626
  Bottom 0.8: 84.6,27.8 84.6,26
S$627
  Bottom 0.8: 81.6,30 81.6,31.8
S$628
  Bottom 0.8: 83.6,30 83.6,31.8
S$629
  Bottom 0.8: 10.2,27.8 10.2,26
S$630
  Bottom 0.8: 12.2,27.8 12.2,26
S$631
  Bottom 0.8: 9.2,30 9.2,31.8
S$632
  Bottom 0.8: 11.2,30 11.2,31.8
S$633
  Bottom 0.8: 6.2,27.8 6.2,26
S$634
  Bottom 0.8: 8.2,27.8 8.2,26
S$635
  Bottom 0.8: 7.2,30 7.2,31.8
S$636
  Bottom 0.8: 5.2,30 5.2,31.8
S$637
  Bottom 0.8: 4.2,27.8 4.2,26
S$638
  Bottom 0.8: 2.2,27.8 2.2,26
S$639
  Bottom 0.8: 3.2,30 3.2,31.8
S$640
  Bottom 0.8: 1.2,30 1.2,31.8
S$641
  Bottom 0.8: 0.2,27.8 0.2,26
S$642
  Bottom 0.8: -1.8,27.8 -1.8,26
S$643
  Bottom 0.8: -0.8,30 -0.8,31.8
S$644
  Bottom 0.8: 18.2,27.8 18.2,26
S$645
  Bottom 0.8: 20.2,27.8 20.2,26
S$646
  Bottom 0.8: 17.2,30 17.2,31.8
S$647
  Bottom 0.8: 19.2,30 19.2,31.8
S$648
  Bottom 0.8: 14.2,27.8 14.2,26
S$649
  Bottom 0.8: 16.2,27.8 16.2,26
S$650
  Bottom 0.8: 13.2,30 13.2,31.8
S$651
  Bottom 0.8: 15.2,30 15.2,31.8
S$652
  Bottom 0.8: 95.8,19.8 95.8,18
S$653
  Bottom 0.8: 97.8,19.8 97.8,18
S$654
  Bottom 0.8: 94.8,22 94.8,23.8
S$655
  Bottom 0.8: 96.8,22 96.8,23.8
S$656
  Bottom 0.8: 91.8,19.8 91.8,18
S$657
  Bottom 0.8: 93.8,19.8 93.8,18
S$658
  Bottom 0.8: 92.8,22 92.8,23.8
S$659
  Bottom 0.8: 90.8,22 90.8,23.8
S$660
  Bottom 0.8: 89.8,19.8 89.8,18
S$661
  Bottom 0.8: 87.8,19.8 87.8,18
S$662
  Bottom 0.8: 88.8,22 88.8,23.8
S$663
  Bottom 0.8: 86.8,22 86.8,23.8
S$664
  Bottom 0.8: 85.8,19.8 85.8,18
S$665
  Bottom 0.8: 83.8,19.8 83.8,18
S$666
  Bottom 0.8: 84.8,22 84.8,23.8
S$667
  Bottom 0.8: 103.8,19.8 103.8,18
S$668
  Bottom 0.8: 105.8,19.8 105.8,18
S$669
  Bottom 0.8: 102.8,22 102.8,23.8
S$670
  Bottom 0.8: 104.8,22 104.8,23.8
S$671
  Bottom 0.8: 99.8,19.8 99.8,18
S$672
  Bottom 0.8: 101.8,19.8 101.8,18
S$673
  Bottom 0.8: 98.8,22 98.8,23.8
S$674
  Bottom 0.8: 100.8,22 100.8,23.8
S$675  (via drill 0.2)
  other vias: 1.2,28.9
S$676  (via drill 0.2)
  other vias: 2.8,28.9
S$677  (via drill 0.2)
  other vias: 4.4,28.9
S$678  (via drill 0.2)
  other vias: 6,28.9
S$679  (via drill 0.2)
  other vias: 7.6,28.9
S$680  (via drill 0.2)
  other vias: 9.2,28.9
S$681  (via drill 0.2)
  other vias: 10.8,28.9
S$682  (via drill 0.2)
  other vias: 12.4,28.9
S$683  (via drill 0.2)
  other vias: 14,28.9
S$684  (via drill 0.2)
  other vias: 15.6,28.9
S$685  (via drill 0.2)
  other vias: 17.2,28.9
S$686  (via drill 0.2)
  other vias: 2,24.9
S$687  (via drill 0.2)
  other vias: 3.6,24.9
S$688  (via drill 0.2)
  other vias: 5.2,24.9
S$689  (via drill 0.2)
  other vias: 6.8,24.9
S$690  (via drill 0.2)
  other vias: 8.4,24.9
S$691  (via drill 0.2)
  other vias: 10,24.9
S$692  (via drill 0.2)
  other vias: 11.6,24.9
S$693  (via drill 0.2)
  other vias: 13.2,24.9
S$694  (via drill 0.2)
  other vias: 14.8,24.9
S$695  (via drill 0.2)
  other vias: 16.4,24.9
S$696  (via drill 0.2)
  other vias: 18,20.9
S$697  (via drill 0.2)
  other vias: 19.6,20.9
S$698  (via drill 0.2)
  other vias: 21.2,20.9
S$699  (via drill 0.2)
  other vias: 22.8,20.9
S$700  (via drill 0.2)
  other vias: 24.4,20.9
S$701  (via drill 0.2)
  other vias: 18.8,24.9
S$702  (via drill 0.2)
  other vias: 20.4,24.9
S$703  (via drill 0.2)
  other vias: 22,24.9
S$704  (via drill 0.2)
  other vias: 23.6,24.9
S$705  (via drill 0.2)
  other vias: 25.2,24.9
S$706  (via drill 0.2)
  other vias: 26,20.9
S$707  (via drill 0.2)
  other vias: 51.6,28.9
S$708  (via drill 0.2)
  other vias: 50,28.9
S$709  (via drill 0.2)
  other vias: 48.4,28.9
S$710  (via drill 0.2)
  other vias: 46.8,28.9
S$711  (via drill 0.2)
  other vias: 45.2,28.9
S$712  (via drill 0.2)
  other vias: 43.6,28.9
S$713  (via drill 0.2)
  other vias: 42,28.9
S$714  (via drill 0.2)
  other vias: 40.4,28.9
S$715  (via drill 0.2)
  other vias: 38.8,28.9
S$716  (via drill 0.2)
  other vias: 37.2,28.9
S$717  (via drill 0.2)
  other vias: 35.6,28.9
S$718  (via drill 0.2)
  other vias: 50.8,24.9
S$719  (via drill 0.2)
  other vias: 49.2,24.9
S$720  (via drill 0.2)
  other vias: 47.6,24.9
S$721  (via drill 0.2)
  other vias: 46,24.9
S$722  (via drill 0.2)
  other vias: 44.4,24.9
S$723  (via drill 0.2)
  other vias: 42.8,24.9
S$724  (via drill 0.2)
  other vias: 41.2,24.9
S$725  (via drill 0.2)
  other vias: 39.6,24.9
S$726  (via drill 0.2)
  other vias: 38,24.9
S$727  (via drill 0.2)
  other vias: 36.4,24.9
S$728  (via drill 0.2)
  other vias: 34.8,20.9
S$729  (via drill 0.2)
  other vias: 33.2,20.9
S$730  (via drill 0.2)
  other vias: 31.6,20.9
S$731  (via drill 0.2)
  other vias: 30,20.9
S$732  (via drill 0.2)
  other vias: 28.4,20.9
S$733  (via drill 0.2)
  other vias: 34,24.9
S$734  (via drill 0.2)
  other vias: 32.4,24.9
S$735  (via drill 0.2)
  other vias: 30.8,24.9
S$736  (via drill 0.2)
  other vias: 29.2,24.9
S$737  (via drill 0.2)
  other vias: 27.6,24.9
S$738  (via drill 0.2)
  other vias: 26.8,20.9
S$739  (via drill 0.2)
  other vias: 52.4,24.9
S$740  (via drill 0.2)
  other vias: 54,24.9
S$741  (via drill 0.2)
  other vias: 55.6,24.9
S$742  (via drill 0.2)
  other vias: 57.2,24.9
S$743  (via drill 0.2)
  other vias: 58.8,24.9
S$744  (via drill 0.2)
  other vias: 60.4,24.9
S$745  (via drill 0.2)
  other vias: 62,24.9
S$746  (via drill 0.2)
  other vias: 63.6,24.9
S$747  (via drill 0.2)
  other vias: 65.2,24.9
S$748  (via drill 0.2)
  other vias: 66.8,24.9
S$749  (via drill 0.2)
  other vias: 68.4,20.9
S$750  (via drill 0.2)
  other vias: 53.2,20.9
S$751  (via drill 0.2)
  other vias: 54.8,20.9
S$752  (via drill 0.2)
  other vias: 56.4,20.9
S$753  (via drill 0.2)
  other vias: 58,20.9
S$754  (via drill 0.2)
  other vias: 59.6,20.9
S$755  (via drill 0.2)
  other vias: 61.2,20.9
S$756  (via drill 0.2)
  other vias: 62.8,20.9
S$757  (via drill 0.2)
  other vias: 64.4,20.9
S$758  (via drill 0.2)
  other vias: 66,20.9
S$759  (via drill 0.2)
  other vias: 67.6,20.9
S$760  (via drill 0.2)
  other vias: 69.2,24.9
S$761  (via drill 0.2)
  other vias: 70.8,24.9
S$762  (via drill 0.2)
  other vias: 72.4,24.9
S$763  (via drill 0.2)
  other vias: 70,28.9
S$764  (via drill 0.2)
  other vias: 71.6,28.9
S$765  (via drill 0.2)
  other vias: 73.2,28.9
S$766  (via drill 0.2)
  other vias: 74,24.9
S$767  (via drill 0.2)
  other vias: 74.8,28.9
S$768  (via drill 0.2)
  other vias: 75.6,24.9
S$769  (via drill 0.2)
  other vias: 76.4,28.9
S$770  (via drill 0.2)
  other vias: 77.2,24.9
S$771  (via drill 0.2)
  other vias: 102.8,24.9
S$772  (via drill 0.2)
  other vias: 101.2,24.9
S$773  (via drill 0.2)
  other vias: 99.6,24.9
S$774  (via drill 0.2)
  other vias: 98,24.9
S$775  (via drill 0.2)
  other vias: 96.4,24.9
S$776  (via drill 0.2)
  other vias: 94.8,24.9
S$777  (via drill 0.2)
  other vias: 93.2,24.9
S$778  (via drill 0.2)
  other vias: 91.6,24.9
S$779  (via drill 0.2)
  other vias: 90,24.9
S$780  (via drill 0.2)
  other vias: 88.4,24.9
S$781  (via drill 0.2)
  other vias: 86.8,20.9
S$782  (via drill 0.2)
  other vias: 102,20.9
S$783  (via drill 0.2)
  other vias: 100.4,20.9
S$784  (via drill 0.2)
  other vias: 98.8,20.9
S$785  (via drill 0.2)
  other vias: 97.2,20.9
S$786  (via drill 0.2)
  other vias: 95.6,20.9
S$787  (via drill 0.2)
  other vias: 94,20.9
S$788  (via drill 0.2)
  other vias: 92.4,20.9
S$789  (via drill 0.2)
  other vias: 90.8,20.9
S$790  (via drill 0.2)
  other vias: 89.2,20.9
S$791  (via drill 0.2)
  other vias: 87.6,20.9
S$792  (via drill 0.2)
  other vias: 86,24.9
S$793  (via drill 0.2)
  other vias: 84.4,24.9
S$794  (via drill 0.2)
  other vias: 82.8,24.9
S$795  (via drill 0.2)
  other vias: 85.2,28.9
S$796  (via drill 0.2)
  other vias: 83.6,28.9
S$797  (via drill 0.2)
  other vias: 82,28.9
S$798  (via drill 0.2)
  other vias: 81.2,24.9
S$799  (via drill 0.2)
  other vias: 80.4,28.9
S$800  (via drill 0.2)
  other vias: 79.6,24.9
S$801  (via drill 0.2)
  other vias: 78.8,28.9
S$802  (via drill 0.2)
  other vias: 78,24.9
S$803
  Bottom 0.152: -0.8,29.9 0.2,28.9
S$804
  Bottom 0.152: 0.2,28.9 1.2,28.9
S$805
  Bottom 0.152: 1.2,29.9 1.8,29.9
S$806
  Bottom 0.152: 1.8,29.9 2.8,28.9
S$807
  Bottom 0.152: 3.2,29.9 3.4,29.9
S$808
  Bottom 0.152: 3.4,29.9 4.4,28.9
S$809
  Bottom 0.152: 5.2,29.9 6,29.1
S$810
  Bottom 0.152: 6,29.1 6,28.9
S$811
  Bottom 0.152: 7.2,29.9 7.6,29.5
S$812
  Bottom 0.152: 7.6,29.5 7.6,28.9
S$813
  Bottom 0.152: 9.2,29.9 9.2,28.9
S$814
  Bottom 0.152: 11.2,29.9 10.8,29.5
S$815
  Bottom 0.152: 10.8,29.5 10.8,28.9
S$816
  Bottom 0.152: 13.2,29.9 12.4,29.1
S$817
  Bottom 0.152: 12.4,29.1 12.4,28.9
S$818
  Bottom 0.152: 15.2,29.9 15,29.9
S$819
  Bottom 0.152: 15,29.9 14,28.9
S$820
  Bottom 0.152: 17.2,29.9 16.6,29.9
S$821
  Bottom 0.152: 16.6,29.9 15.6,28.9
S$822
  Bottom 0.152: 19.2,29.9 18.2,28.9
S$823
  Bottom 0.152: 18.2,28.9 17.2,28.9
S$824
  Bottom 0.152: 0.2,25.9 1.2,24.9
S$825
  Bottom 0.152: 1.2,24.9 2,24.9
S$826
  Bottom 0.152: 2.2,25.9 3.2,24.9
S$827
  Bottom 0.152: 3.2,24.9 3.6,24.9
S$828
  Bottom 0.152: 4.2,25.9 5.2,24.9
S$829
  Bottom 0.152: 6.2,25.9 6.8,25.3
S$830
  Bottom 0.152: 6.8,25.3 6.8,24.9
S$831
  Bottom 0.152: 8.2,25.9 8.4,25.7
S$832
  Bottom 0.152: 8.4,25.7 8.4,24.9
S$833
  Bottom 0.152: 10.2,25.9 10,25.7
S$834
  Bottom 0.152: 10,25.7 10,24.9
S$835
  Bottom 0.152: 12.2,25.9 11.6,25.3
S$836
  Bottom 0.152: 11.6,25.3 11.6,24.9
S$837
  Bottom 0.152: 14.2,25.9 13.2,24.9
S$838
  Bottom 0.152: 16.2,25.9 15.2,24.9
S$839
  Bottom 0.152: 15.2,24.9 14.8,24.9
S$840
  Bottom 0.152: 18.2,25.9 17.2,24.9
S$841
  Bottom 0.152: 17.2,24.9 16.4,24.9
S$842
  Bottom 0.152: 15.4,19.9 16.4,20.9
S$843
  Bottom 0.152: 16.4,20.9 18,20.9
S$844
  Bottom 0.152: 17.4,19.9 18.2,19.9
S$845
  Bottom 0.152: 18.2,19.9 19.2,20.9
S$846
  Bottom 0.152: 19.2,20.9 19.6,20.9
S$847
  Bottom 0.152: 19.4,19.9 20.2,19.9
S$848
  Bottom 0.152: 20.2,19.9 21.2,20.9
S$849
  Bottom 0.152: 21.4,19.9 21.8,19.9
S$850
  Bottom 0.152: 21.8,19.9 22.8,20.9
S$851
  Bottom 0.152: 23.4,19.9 24.4,20.9
S$852
  Bottom 0.152: 25.4,19.9 26,20.5
S$853
  Bottom 0.152: 26,20.5 26,20.9
S$854
  Bottom 0.152: 16.4,23.9 17,23.9
S$855
  Bottom 0.152: 17,23.9 18,24.9
S$856
  Bottom 0.152: 18,24.9 18.8,24.9
S$857
  Bottom 0.152: 18.4,23.9 19,23.9
S$858
  Bottom 0.152: 19,23.9 20,24.9
S$859
  Bottom 0.152: 20,24.9 20.4,24.9
S$860
  Bottom 0.152: 20.4,23.9 21,23.9
S$861
  Bottom 0.152: 21,23.9 22,24.9
S$862
  Bottom 0.152: 22.4,23.9 22.6,23.9
S$863
  Bottom 0.152: 22.6,23.9 23.6,24.9
S$864
  Bottom 0.152: 24.4,23.9 25.2,24.7
S$865
  Bottom 0.152: 25.2,24.7 25.2,24.9
S$866
  Bottom 0.152: 53.6,29.9 52.6,28.9
S$867
  Bottom 0.152: 52.6,28.9 51.6,28.9
S$868
  Bottom 0.152: 51.6,29.9 51,29.9
S$869
  Bottom 0.152: 51,29.9 50,28.9
S$870
  Bottom 0.152: 49.6,29.9 49.4,29.9
S$871
  Bottom 0.152: 49.4,29.9 48.4,28.9
S$872
  Bottom 0.152: 47.6,29.9 46.8,29.1
S$873
  Bottom 0.152: 46.8,29.1 46.8,28.9
S$874
  Bottom 0.152: 45.6,29.9 45.2,29.5
S$875
  Bottom 0.152: 45.2,29.5 45.2,28.9
S$876
  Bottom 0.152: 43.6,29.9 43.6,28.9
S$877
  Bottom 0.152: 41.6,29.9 42,29.5
S$878
  Bottom 0.152: 42,29.5 42,28.9
S$879
  Bottom 0.152: 39.6,29.9 40.4,29.1
S$880
  Bottom 0.152: 40.4,29.1 40.4,28.9
S$881
  Bottom 0.152: 37.6,29.9 37.8,29.9
S$882
  Bottom 0.152: 37.8,29.9 38.8,28.9
S$883
  Bottom 0.152: 35.6,29.9 36.2,29.9
S$884
  Bottom 0.152: 36.2,29.9 37.2,28.9
S$885
  Bottom 0.152: 33.6,29.9 34.6,28.9
S$886
  Bottom 0.152: 34.6,28.9 35.6,28.9
S$887
  Bottom 0.152: 52.6,25.9 51.6,24.9
S$888
  Bottom 0.152: 51.6,24.9 50.8,24.9
S$889
  Bottom 0.152: 50.6,25.9 49.6,24.9
S$890
  Bottom 0.152: 49.6,24.9 49.2,24.9
S$891
  Bottom 0.152: 48.6,25.9 47.6,24.9
S$892
  Bottom 0.152: 46.6,25.9 46,25.3
S$893
  Bottom 0.152: 46,25.3 46,24.9
S$894
  Bottom 0.152: 44.6,25.9 44.4,25.7
S$895
  Bottom 0.152: 44.4,25.7 44.4,24.9
S$896
  Bottom 0.152: 42.6,25.9 42.8,25.7
S$897
  Bottom 0.152: 42.8,25.7 42.8,24.9
S$898
  Bottom 0.152: 40.6,25.9 41.2,25.3
S$899
  Bottom 0.152: 41.2,25.3 41.2,24.9
S$900
  Bottom 0.152: 38.6,25.9 39.6,24.9
S$901
  Bottom 0.152: 36.6,25.9 37.6,24.9
S$902
  Bottom 0.152: 37.6,24.9 38,24.9
S$903
  Bottom 0.152: 34.6,25.9 35.6,24.9
S$904
  Bottom 0.152: 35.6,24.9 36.4,24.9
S$905
  Bottom 0.152: 37.4,19.9 36.4,20.9
S$906
  Bottom 0.152: 36.4,20.9 34.8,20.9
S$907
  Bottom 0.152: 35.4,19.9 34.6,19.9
S$908
  Bottom 0.152: 34.6,19.9 33.6,20.9
S$909
  Bottom 0.152: 33.6,20.9 33.2,20.9
S$910
  Bottom 0.152: 33.4,19.9 32.6,19.9
S$911
  Bottom 0.152: 32.6,19.9 31.6,20.9
S$912
  Bottom 0.152: 31.4,19.9 31,19.9
S$913
  Bottom 0.152: 31,19.9 30,20.9
S$914
  Bottom 0.152: 29.4,19.9 28.4,20.9
S$915
  Bottom 0.152: 27.4,19.9 26.8,20.5
S$916
  Bottom 0.152: 26.8,20.5 26.8,20.9
S$917
  Bottom 0.152: 36.4,23.9 35.8,23.9
S$918
  Bottom 0.152: 35.8,23.9 34.8,24.9
S$919
  Bottom 0.152: 34.8,24.9 34,24.9
S$920
  Bottom 0.152: 34.4,23.9 33.8,23.9
S$921
  Bottom 0.152: 33.8,23.9 32.8,24.9
S$922
  Bottom 0.152: 32.8,24.9 32.4,24.9
S$923
  Bottom 0.152: 32.4,23.9 31.8,23.9
S$924
  Bottom 0.152: 31.8,23.9 30.8,24.9
S$925
  Bottom 0.152: 30.4,23.9 30.2,23.9
S$926
  Bottom 0.152: 30.2,23.9 29.2,24.9
S$927
  Bottom 0.152: 28.4,23.9 27.6,24.7
S$928
  Bottom 0.152: 27.6,24.7 27.6,24.9
S$929
  Bottom 0.152: 52.4,23.9 53,23.9
S$930
  Bottom 0.152: 53,23.9 54,24.9
S$931
  Bottom 0.152: 54.4,23.9 54.6,23.9
S$932
  Bottom 0.152: 54.6,23.9 55.6,24.9
S$933
  Bottom 0.152: 56.4,23.9 57.2,24.7
S$934
  Bottom 0.152: 57.2,24.7 57.2,24.9
S$935
  Bottom 0.152: 58.4,23.9 58.8,24.3
S$936
  Bottom 0.152: 58.8,24.3 58.8,24.9
S$937
  Bottom 0.152: 60.4,23.9 60.4,24.9
S$938
  Bottom 0.152: 50.4,23.9 51.4,23.9
S$939
  Bottom 0.152: 51.4,23.9 52.4,24.9
S$940
  Bottom 0.152: 51.4,19.9 52.4,20.9
S$941
  Bottom 0.152: 52.4,20.9 53.2,20.9
S$942
  Bottom 0.152: 53.4,19.9 53.8,19.9
S$943
  Bottom 0.152: 53.8,19.9 54.8,20.9
S$944
  Bottom 0.152: 55.4,19.9 56.4,20.9
S$945
  Bottom 0.152: 57.4,19.9 58,20.5
S$946
  Bottom 0.152: 58,20.5 58,20.9
S$947
  Bottom 0.152: 59.4,19.9 59.6,20.1
S$948
  Bottom 0.152: 59.6,20.1 59.6,20.9
S$949
  Bottom 0.152: 61.4,19.9 61.2,20.1
S$950
  Bottom 0.152: 61.2,20.1 61.2,20.9
S$951
  Bottom 0.152: 63.4,19.9 62.8,20.5
S$952
  Bottom 0.152: 62.8,20.5 62.8,20.9
S$953
  Bottom 0.152: 65.4,19.9 64.4,20.9
S$954
  Bottom 0.152: 67.4,19.9 67,19.9
S$955
  Bottom 0.152: 67,19.9 66,20.9
S$956
  Bottom 0.152: 69.4,19.9 68.6,19.9
S$957
  Bottom 0.152: 68.6,19.9 67.6,20.9
S$958
  Bottom 0.152: 62.4,23.9 62,24.3
S$959
  Bottom 0.152: 62,24.3 62,24.9
S$960
  Bottom 0.152: 64.4,23.9 63.6,24.7
S$961
  Bottom 0.152: 63.6,24.7 63.6,24.9
S$962
  Bottom 0.152: 66.4,23.9 66.2,23.9
S$963
  Bottom 0.152: 66.2,23.9 65.2,24.9
S$964
  Bottom 0.152: 68.4,23.9 67.8,23.9
S$965
  Bottom 0.152: 67.8,23.9 66.8,24.9
S$966
  Bottom 0.152: 70.4,21.9 69.4,20.9
S$967
  Bottom 0.152: 69.4,20.9 68.4,20.9
S$968
  Bottom 0.152: 68.6,25.9 69.2,25.9
S$969
  Bottom 0.152: 69.2,25.9 70.2,24.9
S$970
  Bottom 0.152: 70.2,24.9 70.8,24.9
S$971
  Bottom 0.152: 70.6,25.9 71.6,24.9
S$972
  Bottom 0.152: 71.6,24.9 72.4,24.9
S$973
  Bottom 0.152: 72.6,25.9 73.6,24.9
S$974
  Bottom 0.152: 73.6,24.9 74,24.9
S$975
  Bottom 0.152: 74.6,25.9 75.6,24.9
S$976
  Bottom 0.152: 76.6,25.9 77.2,25.3
S$977
  Bottom 0.152: 77.2,25.3 77.2,24.9
S$978
  Bottom 0.152: 67.6,29.9 68.6,28.9
S$979
  Bottom 0.152: 68.6,28.9 70,28.9
S$980
  Bottom 0.152: 69.6,29.9 70,29.9
S$981
  Bottom 0.152: 70,29.9 71,28.9
S$982
  Bottom 0.152: 71,28.9 71.6,28.9
S$983
  Bottom 0.152: 71.6,29.9 72.2,29.9
S$984
  Bottom 0.152: 72.2,29.9 73.2,28.9
S$985
  Bottom 0.152: 73.6,29.9 73.8,29.9
S$986
  Bottom 0.152: 73.8,29.9 74.8,28.9
S$987
  Bottom 0.152: 75.6,29.9 76.4,29.1
S$988
  Bottom 0.152: 76.4,29.1 76.4,28.9
S$989
  Bottom 0.152: 69.2,24.9 68,24.9
S$990
  Bottom 0.152: 68,24.9 67,25.9
S$991
  Top 1.778: -51.08,3.73 -51.08,5.25
S$992
  Top 1.778: -46,3.73 -46,5.25
S$993
  Top 1.778: -40.92,3.73 -40.92,5.25
S$994
  Bottom 0.152: 67,25.9 66.6,25.9
S$995
  Bottom 0.152: 102.8,23.9 102.2,23.9
S$996
  Bottom 0.152: 102.2,23.9 101.2,24.9
S$997
  Bottom 0.152: 100.8,23.9 100.6,23.9
S$998
  Bottom 0.152: 100.6,23.9 99.6,24.9
S$999
  Bottom 0.152: 98.8,23.9 98,24.7
S$1000
  Bottom 0.152: 98,24.7 98,24.9
S$1001
  Bottom 0.152: 96.8,23.9 96.4,24.3
S$1002
  Bottom 0.152: 96.4,24.3 96.4,24.9
S$1003
  Bottom 0.152: 94.8,23.9 94.8,24.9
S$1004
  Bottom 0.152: 104.8,23.9 103.8,23.9
S$1005
  Bottom 0.152: 103.8,23.9 102.8,24.9
S$1006
  Bottom 0.152: 103.8,19.9 102.8,20.9
S$1007
  Bottom 0.152: 102.8,20.9 102,20.9
S$1008
  Bottom 0.152: 101.8,19.9 101.4,19.9
S$1009
  Bottom 0.152: 101.4,19.9 100.4,20.9
S$1010
  Bottom 0.152: 99.8,19.9 98.8,20.9
S$1011
  Bottom 0.152: 97.8,19.9 97.2,20.5
S$1012
  Bottom 0.152: 97.2,20.5 97.2,20.9
S$1013
  Bottom 0.152: 95.8,19.9 95.6,20.1
S$1014
  Bottom 0.152: 95.6,20.1 95.6,20.9
S$1015
  Bottom 0.152: 93.8,19.9 94,20.1
S$1016
  Bottom 0.152: 94,20.1 94,20.9
S$1017
  Bottom 0.152: 91.8,19.9 92.4,20.5
S$1018
  Bottom 0.152: 92.4,20.5 92.4,20.9
S$1019
  Bottom 0.152: 89.8,19.9 90.8,20.9
S$1020
  Bottom 0.152: 87.8,19.9 88.2,19.9
S$1021
  Bottom 0.152: 88.2,19.9 89.2,20.9
S$1022
  Bottom 0.152: 85.8,19.9 86.6,19.9
S$1023
  Bottom 0.152: 86.6,19.9 87.6,20.9
S$1024
  Bottom 0.152: 92.8,23.9 93.2,24.3
S$1025
  Bottom 0.152: 93.2,24.3 93.2,24.9
S$1026
  Bottom 0.152: 90.8,23.9 91.6,24.7
S$1027
  Bottom 0.152: 91.6,24.7 91.6,24.9
S$1028
  Bottom 0.152: 88.8,23.9 89,23.9
S$1029
  Bottom 0.152: 89,23.9 90,24.9
S$1030
  Bottom 0.152: 86.8,23.9 87.4,23.9
S$1031
  Bottom 0.152: 87.4,23.9 88.4,24.9
S$1032
  Bottom 0.152: 84.8,21.9 85.8,20.9
S$1033
  Bottom 0.152: 85.8,20.9 86.8,20.9
S$1034
  Bottom 0.152: 86.6,25.9 86,25.9
S$1035
  Bottom 0.152: 86,25.9 85,24.9
S$1036
  Bottom 0.152: 85,24.9 84.4,24.9
S$1037
  Bottom 0.152: 84.6,25.9 83.6,24.9
S$1038
  Bottom 0.152: 83.6,24.9 82.8,24.9
S$1039
  Bottom 0.152: 82.6,25.9 81.6,24.9
S$1040
  Bottom 0.152: 81.6,24.9 81.2,24.9
S$1041
  Bottom 0.152: 80.6,25.9 79.6,24.9
S$1042
  Bottom 0.152: 78.6,25.9 78,25.3
S$1043
  Bottom 0.152: 78,25.3 78,24.9
S$1044
  Bottom 0.152: 87.6,29.9 86.6,28.9
S$1045
  Bottom 0.152: 86.6,28.9 85.2,28.9
S$1046
  Bottom 0.152: 85.6,29.9 85.2,29.9
S$1047
  Bottom 0.152: 85.2,29.9 84.2,28.9
S$1048
  Bottom 0.152: 84.2,28.9 83.6,28.9
S$1049
  Bottom 0.152: 83.6,29.9 83,29.9
S$1050
  Bottom 0.152: 83,29.9 82,28.9
S$1051
  Bottom 0.152: 81.6,29.9 81.4,29.9
S$1052
  Bottom 0.152: 81.4,29.9 80.4,28.9
S$1053
  Bottom 0.152: 79.6,29.9 78.8,29.1
S$1054
  Bottom 0.152: 78.8,29.1 78.8,28.9
S$1055
  Bottom 0.152: 86,24.9 87.2,24.9
S$1056
  Bottom 0.152: 87.2,24.9 88.2,25.9
S$1057
  Bottom 0.152: 88.2,25.9 88.6,25.9
S$1058  (4 unrouted)
  Top 0.508: -13,27.9 -13,23.4 | -13,23.4 -13,21.9 | -13,23.4 -16.5,23.4 -18,24.9 -41,24.9 -41,23.4 -41,25.9 | 117,29.4 117,24.9 | 117,24.9 117,20.4 | 117,24.9 145,24.9 145,26.9
  Top 1.8: -12,24.9 -14,24.9 | -12,27.9 -13,27.9 -14,27.9 | -12,21.9 -13,21.9 -14,21.9 | 118,26.4 116,26.4 | 118,29.4 117,29.4 116,29.4 | 118,23.4 116,23.4 | 118,20.4 117,20.4 116,20.4
S$1059
  Top 1.778: -51.08,21.73 -51.08,23.25
S$1060
  Top 1.778: -51.08,26.55 -51.08,28.08
S$1061
  Top 1.778: -46,21.73 -46,23.25
S$1062
  Top 1.778: -46,26.55 -46,28.08
S$1063
  Top 1.778: -40.92,21.73 -40.92,23.25
S$1064
  Top 1.778: -40.92,26.55 -40.92,28.08
S$1065
  Top 1.778: 144.92,21.73 144.92,23.25
S$1066
  Top 1.778: 144.92,26.55 144.92,28.08
S$1067
  Top 1.778: 150,21.73 150,23.25
S$1068
  Top 1.778: 150,26.55 150,28.08
S$1069
  Top 1.778: 155.08,21.73 155.08,23.25
S$1070
  Top 1.778: 155.08,26.55 155.08,28.08
S$1071  (via drill 0.2)
  other vias: 26.4,31.3
S$1072  (via drill 0.2)
  other vias: 43.4,18.5
S$1073  (via drill 0.2)
  other vias: 60.6,31.3
S$1074  (via drill 0.2)
  other vias: 77.6,18.5
S$1075  (via drill 0.2)
  other vias: 93.6,31.3
S$1076  (via drill 0.2)
  other vias: 104.8,31.3
S$1077  (via drill 0.2)
  other vias: 10.4,18.5
S$1078  (via drill 0.2)
  other vias: -0.8,18.5
S$1079
  Bottom 0.8: 61.4,37.8 61.4,36
S$1080
  Bottom 0.8: 63.4,37.8 63.4,36
S$1081
  Bottom 0.8: 60.4,40 60.4,41.8
S$1082
  Bottom 0.8: 62.4,40 62.4,41.8
S$1083
  Bottom 0.8: 57.4,37.8 57.4,36
S$1084
  Bottom 0.8: 59.4,37.8 59.4,36
S$1085
  Bottom 0.8: 58.4,40 58.4,41.8
S$1086
  Bottom 0.8: 56.4,40 56.4,41.8
S$1087
  Bottom 0.8: 55.4,37.8 55.4,36
S$1088
  Bottom 0.8: 53.4,37.8 53.4,36
S$1089
  Bottom 0.8: 54.4,40 54.4,41.8
S$1090
  Bottom 0.8: 52.4,40 52.4,41.8
S$1091
  Bottom 0.8: 51.4,37.8 51.4,36
S$1092
  Bottom 0.8: 49.4,37.8 49.4,36
S$1093
  Bottom 0.8: 50.4,40 50.4,41.8
S$1094
  Bottom 0.8: 69.4,37.8 69.4,36
S$1095
  Bottom 0.8: 71.4,37.8 71.4,36
S$1096
  Bottom 0.8: 68.4,40 68.4,41.8
S$1097
  Bottom 0.8: 70.4,40 70.4,41.8
S$1098
  Bottom 0.8: 65.4,37.8 65.4,36
S$1099
  Bottom 0.8: 67.4,37.8 67.4,36
S$1100
  Bottom 0.8: 64.4,40 64.4,41.8
S$1101
  Bottom 0.8: 66.4,40 66.4,41.8
S$1102
  Bottom 0.8: 44.6,45.8 44.6,44
S$1103
  Bottom 0.8: 46.6,45.8 46.6,44
S$1104
  Bottom 0.8: 43.6,48 43.6,49.8
S$1105
  Bottom 0.8: 45.6,48 45.6,49.8
S$1106
  Bottom 0.8: 40.6,45.8 40.6,44
S$1107
  Bottom 0.8: 42.6,45.8 42.6,44
S$1108
  Bottom 0.8: 41.6,48 41.6,49.8
S$1109
  Bottom 0.8: 39.6,48 39.6,49.8
S$1110
  Bottom 0.8: 38.6,45.8 38.6,44
S$1111
  Bottom 0.8: 36.6,45.8 36.6,44
S$1112
  Bottom 0.8: 37.6,48 37.6,49.8
S$1113
  Bottom 0.8: 35.6,48 35.6,49.8
S$1114
  Bottom 0.8: 34.6,45.8 34.6,44
S$1115
  Bottom 0.8: 32.6,45.8 32.6,44
S$1116
  Bottom 0.8: 33.6,48 33.6,49.8
S$1117
  Bottom 0.8: 52.6,45.8 52.6,44
S$1118
  Bottom 0.8: 54.6,45.8 54.6,44
S$1119
  Bottom 0.8: 51.6,48 51.6,49.8
S$1120
  Bottom 0.8: 53.6,48 53.6,49.8
S$1121
  Bottom 0.8: 48.6,45.8 48.6,44
S$1122
  Bottom 0.8: 50.6,45.8 50.6,44
S$1123
  Bottom 0.8: 47.6,48 47.6,49.8
S$1124
  Bottom 0.8: 49.6,48 49.6,49.8
S$1125
  Bottom 0.8: 27.4,37.8 27.4,36
S$1126
  Bottom 0.8: 29.4,37.8 29.4,36
S$1127
  Bottom 0.8: 26.4,40 26.4,41.8
S$1128
  Bottom 0.8: 28.4,40 28.4,41.8
S$1129
  Bottom 0.8: 23.4,37.8 23.4,36
S$1130
  Bottom 0.8: 25.4,37.8 25.4,36
S$1131
  Bottom 0.8: 24.4,40 24.4,41.8
S$1132
  Bottom 0.8: 22.4,40 22.4,41.8
S$1133
  Bottom 0.8: 21.4,37.8 21.4,36
S$1134
  Bottom 0.8: 19.4,37.8 19.4,36
S$1135
  Bottom 0.8: 20.4,40 20.4,41.8
S$1136
  Bottom 0.8: 18.4,40 18.4,41.8
S$1137
  Bottom 0.8: 17.4,37.8 17.4,36
S$1138
  Bottom 0.8: 15.4,37.8 15.4,36
S$1139
  Bottom 0.8: 16.4,40 16.4,41.8
S$1140
  Bottom 0.8: 35.4,37.8 35.4,36
S$1141
  Bottom 0.8: 37.4,37.8 37.4,36
S$1142
  Bottom 0.8: 34.4,40 34.4,41.8
S$1143
  Bottom 0.8: 36.4,40 36.4,41.8
S$1144
  Bottom 0.8: 31.4,37.8 31.4,36
S$1145
  Bottom 0.8: 33.4,37.8 33.4,36
S$1146
  Bottom 0.8: 30.4,40 30.4,41.8
S$1147
  Bottom 0.8: 32.4,40 32.4,41.8
S$1148
  Bottom 0.8: 78.6,45.8 78.6,44
S$1149
  Bottom 0.8: 80.6,45.8 80.6,44
S$1150
  Bottom 0.8: 77.6,48 77.6,49.8
S$1151
  Bottom 0.8: 79.6,48 79.6,49.8
S$1152
  Bottom 0.8: 74.6,45.8 74.6,44
S$1153
  Bottom 0.8: 76.6,45.8 76.6,44
S$1154
  Bottom 0.8: 75.6,48 75.6,49.8
S$1155
  Bottom 0.8: 73.6,48 73.6,49.8
S$1156
  Bottom 0.8: 72.6,45.8 72.6,44
S$1157
  Bottom 0.8: 70.6,45.8 70.6,44
S$1158
  Bottom 0.8: 71.6,48 71.6,49.8
S$1159
  Bottom 0.8: 69.6,48 69.6,49.8
S$1160
  Bottom 0.8: 68.6,45.8 68.6,44
S$1161
  Bottom 0.8: 66.6,45.8 66.6,44
S$1162
  Bottom 0.8: 67.6,48 67.6,49.8
S$1163
  Bottom 0.8: 86.6,45.8 86.6,44
S$1164
  Bottom 0.8: 88.6,45.8 88.6,44
S$1165
  Bottom 0.8: 85.6,48 85.6,49.8
S$1166
  Bottom 0.8: 87.6,48 87.6,49.8
S$1167
  Bottom 0.8: 82.6,45.8 82.6,44
S$1168
  Bottom 0.8: 84.6,45.8 84.6,44
S$1169
  Bottom 0.8: 81.6,48 81.6,49.8
S$1170
  Bottom 0.8: 83.6,48 83.6,49.8
S$1171
  Bottom 0.8: 10.2,45.8 10.2,44
S$1172
  Bottom 0.8: 12.2,45.8 12.2,44
S$1173
  Bottom 0.8: 9.2,48 9.2,49.8
S$1174
  Bottom 0.8: 11.2,48 11.2,49.8
S$1175
  Bottom 0.8: 6.2,45.8 6.2,44
S$1176
  Bottom 0.8: 8.2,45.8 8.2,44
S$1177
  Bottom 0.8: 7.2,48 7.2,49.8
S$1178
  Bottom 0.8: 5.2,48 5.2,49.8
S$1179
  Bottom 0.8: 4.2,45.8 4.2,44
S$1180
  Bottom 0.8: 2.2,45.8 2.2,44
S$1181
